(* Logix 5000 AddOnInstructionDefinition export Banner_Q90R2KU_Param_v4; software revision 33.00 *)

TYPE Banner_IOL_Port_v4 :   // UDT that has all of the data items necessary to communicate with a specific Port on a IO-Link Master
STRUCT
   Port_Controlled : INT;   // Each bit represents a port on an IO-Link Master. Set to 1 to tell AOI to control that port.
   Port_Activate : INT;   // Each bit represents a port on an IO-Link Master. When ON that port will process any commands in queue.
   Port_Read : INT;   // Each bit represents a port on an IO-Link Master. Used to determine when device AOI has requested a Read command.
   Port_Write : INT;   // Each bit represents a port on an IO-Link Master. Used to determine when device AOI has requested a Write command.
   Port_RW_Complete : INT;   // Each bit represents a port on an IO-Link Master. Tells device AOI that Read or Write request has been completed.
   Port_Device_Read : INT;
   Data_Transfer : SINT[190];   // Array to transfer data from IO-Master to device AOIs.
END_STRUCT
END_TYPE

TYPE Banner_Q90R2KR_AO1_Config_v4 :
STRUCT
   Output_Type : INT;   // 0=4-20mA, 128=0-10V, 129=0.5-4.5V.
   Measurement : SINT;   // 0=Distance or Y, 1=Velocity
   Loss_of_Signal : SINT;   // 0=Hold, 1=Low, 2=High
   Average : INT;   // 0=1, 1=2, 2=4, 3=8, 4=16, 5=32, 6=64, 7=128
END_STRUCT
END_TYPE

TYPE Banner_Q90R2KU_ActiveSensingRange :
STRUCT
   Detection_Area : SINT;   // 0=Radial, 1=Rectangular
   Radial_Min_Active_Sensing_Distance : DINT;
   Radial_Max_Active_Sensing_Distance : DINT;
   Rectangular_Min_Active_Sensing_Y : DINT;
   Rectangular_Max_Active_Sensing_Y : DINT;
   Velocity_Filter : INT;   // 0=All target velocities, 1=Dynamic targets only, 2=Approaching targets only, 3=Receding targets only, 4=custom
   Min_Velocity : DINT;
   Max_Velocity : DINT;
   Velocity_Hysteresis : DINT;
END_STRUCT
END_TYPE

TYPE Banner_Q90R2KU_AO1_Detection_Area :
STRUCT
   Peak_Select_Mode : SINT;   // 0=First Peak, 1=Strongest Peak
   Radial_Beam_Angle_SP1 : INT;
   Radial_Beam_Angle_SP2 : INT;
   Radial_Beam_Angle_Hysteresis : INT;
   Rectangular_X_SP1 : DINT;
   Rectangular_X_SP2 : DINT;
   Rectangular_X_Hysteresis : DINT;
END_STRUCT
END_TYPE

TYPE Banner_Q90R2KU_AO1_Setpoints_v4 :
STRUCT
   Radial_Distance_SP1 : DINT;
   Radial_Distance_SP2 : DINT;
   Rectangular_Y_SP1 : DINT;
   Rectangular_Y_SP2 : DINT;
   Velocity_SP1 : DINT;
   Velocity_SP2 : DINT;
END_STRUCT
END_TYPE

TYPE Banner_Q90R2KU_Config_v4 :
STRUCT
   Response_Speed : SINT;   // 0 = Fast, 1 = Medium, 2 = Slow
   Detection_Sensitivity : SINT;   // 0=High, 1=Standard
   LEDs_Disabled : SINT;   // 0=Enabled, 1=Standard
   Output_Polarity : SINT;   // 0=NPN, 1=PNP
   PD_Measurement : SINT;   // 0=Radial, 1=Rectangular
   Remote_Input_Mode : SINT;   // 0=Disabled, 1=Teach
   Amplitude_Threshold : DINT;   // 100 to 100000
   Limit_Filter_Enabled : SINT;   // 0=Disabled, 1=Enabled
   Limit_Filter_Positive_Hold_Time : DINT;   // 50 to 3600000
   Limit_Filter_Negative_Hold_Time : DINT;   // 50 to 3600000
   Limit_Filter_Positive_Distance : DINT;   // 0 to 1000
   Limit_Filter_Negative_Distance : DINT;   // 0 to 1000
   Primary_Output_Mode : SINT;   // 0=Independent Output, 1=Complementary Output, 2=Pulse Frequency Output
END_STRUCT
END_TYPE

TYPE Banner_Q90R2KU_Detection_Area :
STRUCT
   Peak_Select_Mode : SINT;   // 0=First Peak, 1=Strongest Peak
   Radial_Beam_Angle_SP1 : INT;
   Radial_Beam_Angle_SP2 : INT;
   Radial_Beam_Angle_Hysteresis : INT;
   Rectangular_X_SP1 : DINT;
   Rectangular_X_SP2 : DINT;
   Rectangular_X_Hysteresis : DINT;
END_STRUCT
END_TYPE

TYPE Banner_Q90R2KU_Direct_v4 :
STRUCT
   Master_Cycle_Time : INT;
   Min_Cycle_Time : INT;
   M_Sequence_Capability : INT;
   IO_Link_Version_ID : INT;
   Process_Data_Input_Length : INT;
   Process_Data_Output_Length : INT;
   Combined_Vendor_ID : DINT;   // IO-Link Vendor ID
   Vendor_ID1 : INT;
   Vendor_ID2 : INT;
   Combined_Device_ID : DINT;   // IO-Link Device ID
   Device_ID1 : INT;
   Device_ID2 : INT;
   Device_ID3 : INT;
END_STRUCT
END_TYPE

TYPE Banner_Q90R2KU_Pulse :
STRUCT
   Measurement : SINT;   // 0=Distance, 1=Velocity
   Frequency_SP1 : DINT;   // 100 to 600 Hz
   Frequency_SP2 : DINT;   // 100 to 600 Hz
   Loss_of_Signal : SINT;   // 0=Hold, 1=Low, 2=High
   Radial_Distance_SP1 : DINT;
   Radial_Distance_SP2 : DINT;
   Rectangular_Y_SP1 : DINT;
   Rectangular_Y_SP2 : DINT;
   Velocity_SP1 : DINT;
   Velocity_SP2 : DINT;
END_STRUCT
END_TYPE

TYPE Banner_Q90R2KU_RD_v4 :   // UDT that stores the Read Data for a Q90R Analog.
STRUCT
   Direct : Banner_Q90R2KU_Direct_v4;
   Serial_Number : STRING;
   Teach_State : SINT;
   SP1_TP1 : SINT;
   SP1_TP2 : SINT;
   SP2_TP1 : SINT;
   SP2_TP2 : SINT;
   Status : Banner_Q90R2KU_Status_v4;
   All_Time_Run_Time : DINT;   // Read only counter that tracks the total time sensor has been running since manufacture. Value in Hours.
END_STRUCT
END_TYPE

TYPE Banner_Q90R2KU_SSC1_Configuration :
STRUCT
   Switch_Point_Logic : SINT;   // 0=LO, 1=DO
   Distance_or_Y_Setpoint_Mode : SINT;   // 1=Switch Mode/Single Point Mode, 2=Window Mode
END_STRUCT
END_TYPE

TYPE Banner_Q90R2KU_SSC1_Setpoints :
STRUCT
   Radial_Distance_SP1 : DINT;
   Radial_Distance_SP2 : DINT;
   Radial_Distance_Hysteresis : DINT;
   Rectangular_Y_SP1 : DINT;
   Rectangular_Y_SP2 : DINT;
   Rectangular_Y_Hysteresis : DINT;
END_STRUCT
END_TYPE

TYPE Banner_Q90R2KU_Status_v4 :
STRUCT
   SSC1_State : SINT;   // 0=Inactive, 1=Active
   SSC1_Stability : SINT;   // 0=No target, 1=Marginal target, 2=Strong target
   SSC1_Distance_or_X : DINT;
   SSC1_Beam_Angle_or_Y : DINT;
   SSC1_Velocity : DINT;
   SSC1_Signal_Strength : INT;
   AO1_State : SINT;   // 0=Inactive, 1=Active
   AO1_Stability : SINT;   // 0=No target, 1=Marginal target, 2=Strong target
   AO1_Distance_or_X : DINT;
   AO1_Beam_Angle_or_Y : DINT;
   AO1_Velocity : DINT;
   AO1_Signal_Strength : INT;
   Fault_Status : SINT;   // 0=No fault present, 1=fault present
   Analog_Output_Value : DINT;
   Temperature : DINT;
   Last_Taught_Temperature : DINT;
END_STRUCT
END_TYPE

TYPE Banner_Q90R2KU_v4 :   // All of the parameters for a Q90R2 Analog.
STRUCT
   Initial_Global_Read : BOOL;   // Determines if all of the IO-Link data has been read into the PLC yet
   Command : INT;   // Value placed in here will activate a read or write to a specifc IO-Link Index
   Read : Banner_Q90R2KU_RD_v4;   // Read Only Data
   Write : Banner_Q90R2KU_WD_v4;   // Write Data
   Archive : Banner_Q90R2KU_WD_v4;   // Archive Data
   Reset : BOOL;   // Resets AOI. This will force a complete parameter read of the sensor.
END_STRUCT
END_TYPE

TYPE Banner_Q90R2KU_Vendor_Specific_Config_v4 :
STRUCT
   Delay_On : DINT;
   Delay_Off : DINT;
   Radial_Distance_Window_Size : DINT;   // This will set the size of the distance window after a teach.
   Radial_Distance_User_Teach_Offset : DINT;   // Distance offset applied to taught switch position.
   Radial_Reserved_Window_Size : DINT;   // This will set the size of the beam-angle window after a teach.
   Radial_Reserved_User_Teach_Offset : DINT;
   Rectangular_Reserved_Window_Size : DINT;
   Rectangular_Reserved_User_Teach_Offset : DINT;
   Rectangular_Y_Window_Size : DINT;
   Rectangular_Y_User_Teach_Offset : DINT;
END_STRUCT
END_TYPE

TYPE Banner_Q90R2KU_WD_v4 :   // UDT that stores the Write Data for a Q90R2KU.
STRUCT
   System_Command : INT;   // See IODD file for list of commands that can be activated via the System Command interface
   Teach_Selection : SINT;   // 0 = Default, 1 = BDC1, 192 = AO1
   Config : Banner_Q90R2KU_Config_v4;
   SSC1_Vendor_Config : Banner_Q90R2KU_Vendor_Specific_Config_v4;
   Resettable_Run_Time : DINT;
   AO1_Setpoints : Banner_Q90R2KU_AO1_Setpoints_v4;
   AO1_Config : Banner_Q90R2KR_AO1_Config_v4;
   All_Time_Run_Time_Event_Time : DINT;
   Resettable_Run_Time_Event_Time : DINT;
   Active_Sensing_Range : Banner_Q90R2KU_ActiveSensingRange;
   SSC1_Config : Banner_Q90R2KU_SSC1_Configuration;
   SSC1_Setpoints : Banner_Q90R2KU_SSC1_Setpoints;
   SSC1_Detection : Banner_Q90R2KU_Detection_Area;
   AO1_Detection : Banner_Q90R2KU_AO1_Detection_Area;
   Pulse : Banner_Q90R2KU_Pulse;
END_STRUCT
END_TYPE

ADD_ON_INSTRUCTION Banner_Q90R2KU_Param_v4   (* revision 4.1, vendor Banner Engineering *)
// AOI to read and write parameter data to an IO-Link Q90R2 Analog.
VAR_IN_OUT
   Q90RKU : Banner_Q90R2KU_v4; {required}
   Port_Data : Banner_IOL_Port_v4; {required}
END_VAR
VAR_INPUT
   Port : DINT; {required}
END_VAR
VAR
   Local_Control : DINT; {access None}
   Global_Read_Command_Value : INT; {access None}
   Global_Write_Command_Value : INT; {access None}
   Command_Being_Processed : BOOL; {access None}
   Update_Archive : BOOL; {access None}
   Index_Write_Inprocess : DINT; {access None}
   Index_Write_Control : DINT; {access None}
   Inprocess_Index : DINT; {access None}
END_VAR

ROUTINE Logic   (* ladder *)
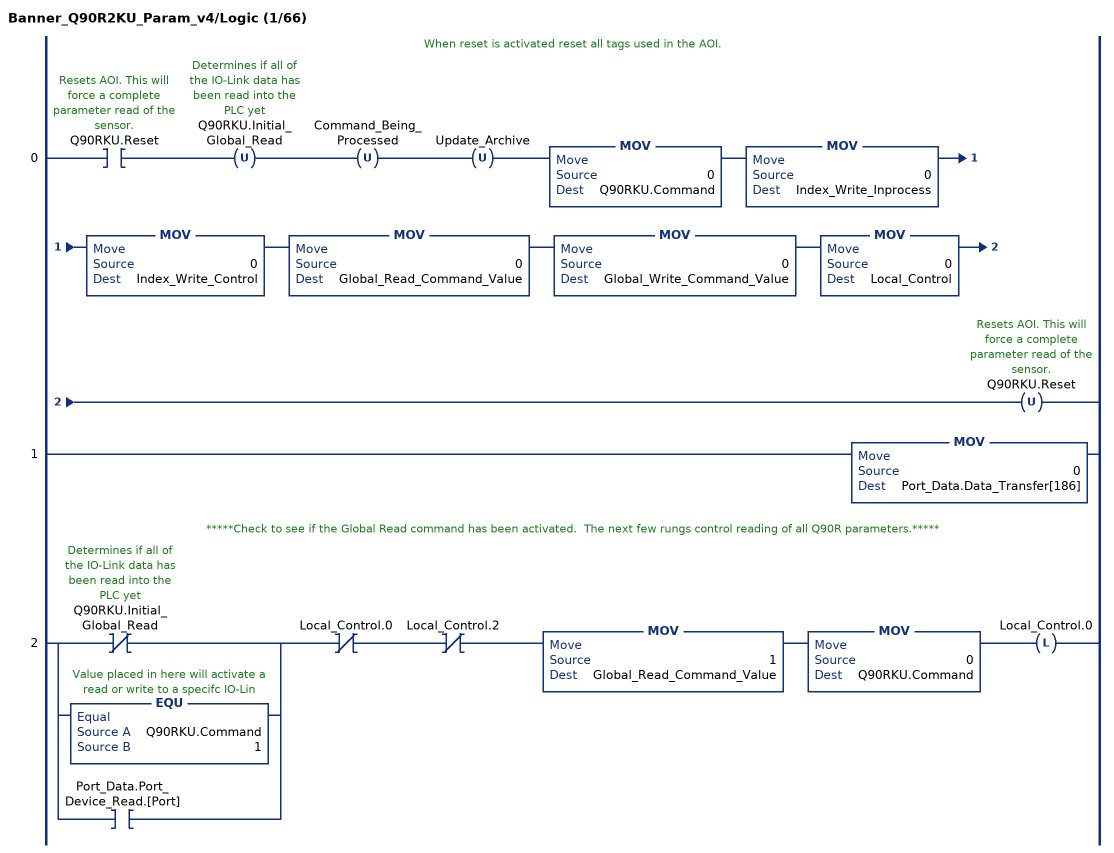
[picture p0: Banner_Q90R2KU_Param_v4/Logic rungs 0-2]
   // When reset is activated reset all tags used in the AOI.
   0: XIC(Q90RKU.Reset)OTU(Q90RKU.Initial_Global_Read)OTU(Command_Being_Processed)OTU(Update_Archive)MOV(0,Q90RKU.Command)MOV(0,Index_Write_Inprocess)MOV(0,Index_Write_Control)MOV(0,Global_Read_Command_Value)MOV(0,Global_Write_Command_Value)MOV(0,Local_Control)OTU(Q90RKU.Reset);
   1: MOV(0,Port_Data.Data_Transfer[186]);
   // *****Check to see if the Global Read command has been activated.  The next few rungs control reading of all Q90R parameters.*****
   2: [XIO(Q90RKU.Initial_Global_Read) ,EQU(Q90RKU.Command,1) ,XIC(Port_Data.Port_Device_Read.[Port]) ]XIO(Local_Control.0)XIO(Local_Control.2)MOV(1,Global_Read_Command_Value)MOV(0,Q90RKU.Command)OTL(Local_Control.0);
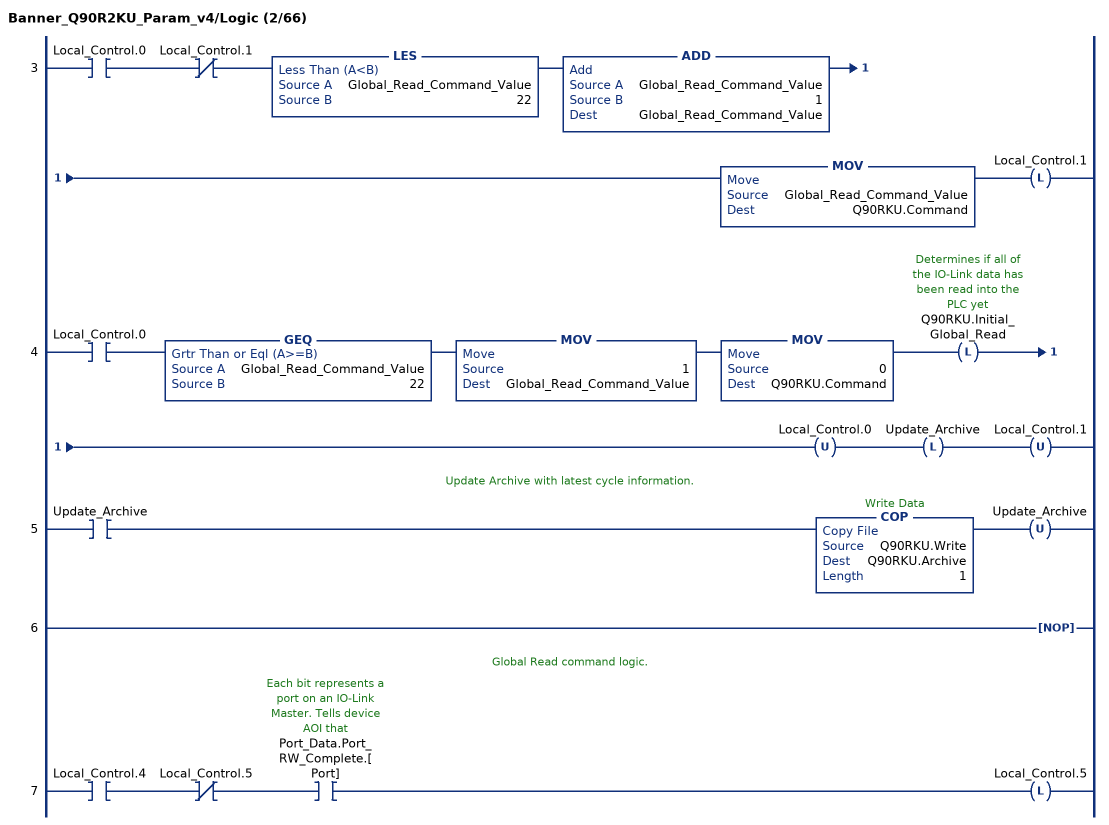
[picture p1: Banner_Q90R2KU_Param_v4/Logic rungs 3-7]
   3: XIC(Local_Control.0)XIO(Local_Control.1)LES(Global_Read_Command_Value,22)ADD(Global_Read_Command_Value,1,Global_Read_Command_Value)MOV(Global_Read_Command_Value,Q90RKU.Command)OTL(Local_Control.1);
   4: XIC(Local_Control.0)GEQ(Global_Read_Command_Value,22)MOV(1,Global_Read_Command_Value)MOV(0,Q90RKU.Command)OTL(Q90RKU.Initial_Global_Read)OTU(Local_Control.0)OTL(Update_Archive)OTU(Local_Control.1);
   // Update Archive with latest cycle information.
   5: XIC(Update_Archive)COP(Q90RKU.Write,Q90RKU.Archive,1)OTU(Update_Archive);
   6: NOP();
   // Global Read command logic.
   7: XIC(Local_Control.4)XIO(Local_Control.5)XIC(Port_Data.Port_RW_Complete.[Port])OTL(Local_Control.5);
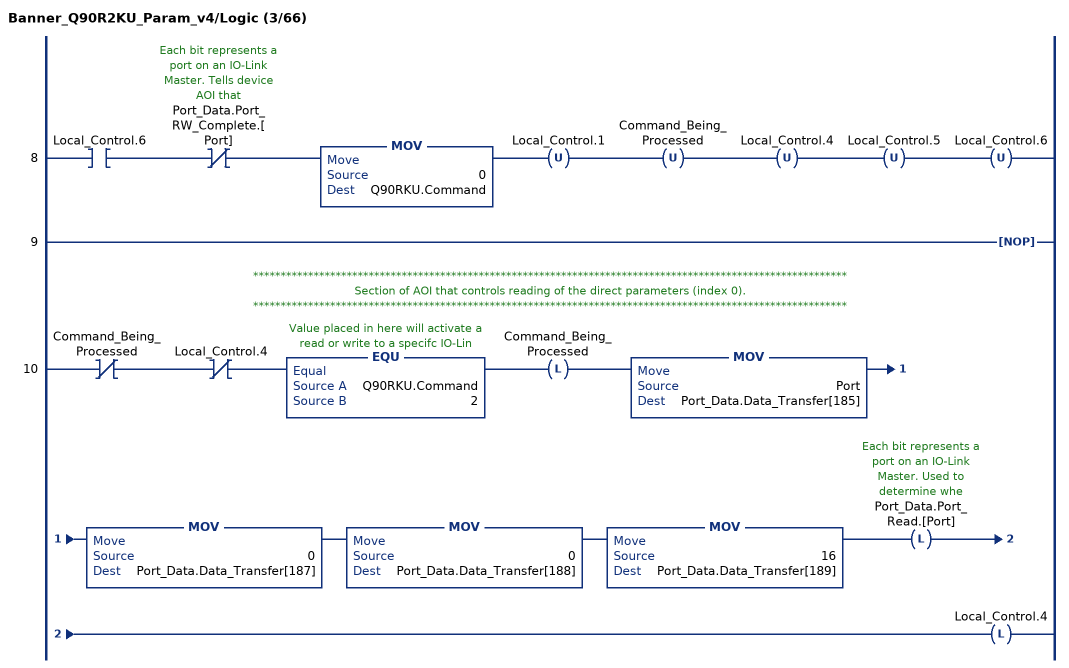
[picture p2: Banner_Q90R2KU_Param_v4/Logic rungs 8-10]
   8: XIC(Local_Control.6)XIO(Port_Data.Port_RW_Complete.[Port])MOV(0,Q90RKU.Command)OTU(Local_Control.1)OTU(Command_Being_Processed)OTU(Local_Control.4)OTU(Local_Control.5)OTU(Local_Control.6);
   9: NOP();
   // ************************************************************************************************************
   // Section of AOI that controls reading of the direct parameters (index 0).
   // ************************************************************************************************************
   10: XIO(Command_Being_Processed)XIO(Local_Control.4)EQU(Q90RKU.Command,2)OTL(Command_Being_Processed)MOV(Port,Port_Data.Data_Transfer[185])MOV(0,Port_Data.Data_Transfer[187])MOV(0,Port_Data.Data_Transfer[188])MOV(16,Port_Data.Data_Transfer[189])OTL(Port_Data.Port_Read.[Port])OTL(Local_Control.4);
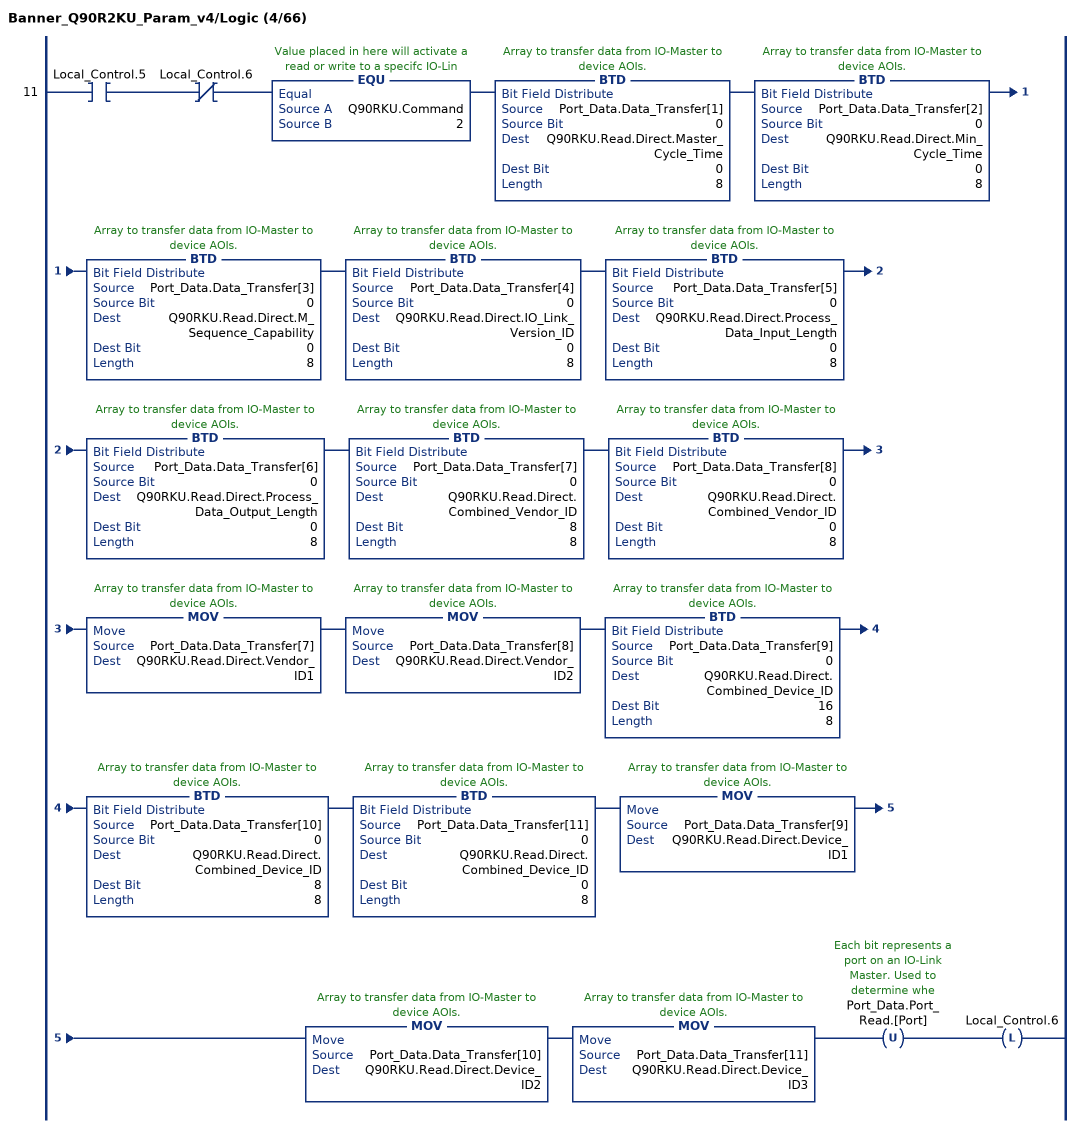
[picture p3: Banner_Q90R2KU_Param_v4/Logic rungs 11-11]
   11: XIC(Local_Control.5)XIO(Local_Control.6)EQU(Q90RKU.Command,2)BTD(Port_Data.Data_Transfer[1],0,Q90RKU.Read.Direct.Master_Cycle_Time,0,8)BTD(Port_Data.Data_Transfer[2],0,Q90RKU.Read.Direct.Min_Cycle_Time,0,8)BTD(Port_Data.Data_Transfer[3],0,Q90RKU.Read.Direct.M_Sequence_Capability,0,8)BTD(Port_Data.Data_Transfer[4],0,Q90RKU.Read.Direct.IO_Link_Version_ID,0,8)BTD(Port_Data.Data_Transfer[5],0,Q90RKU.Read.Direct.Process_Data_Input_Length,0,8)BTD(Port_Data.Data_Transfer[6],0,Q90RKU.Read.Direct.Process_Data_Output_Length,0,8)BTD(Port_Data.Data_Transfer[7],0,Q90RKU.Read.Direct.Combined_Vendor_ID,8,8)BTD(Port_Data.Data_Transfer[8],0,Q90RKU.Read.Direct.Combined_Vendor_ID,0,8)MOV(Port_Data.Data_Transfer[7],Q90RKU.Read.Direct.Vendor_ID1)MOV(Port_Data.Data_Transfer[8],Q90RKU.Read.Direct.Vendor_ID2)BTD(Port_Data.Data_Transfer[9],0,Q90RKU.Read.Direct.Combined_Device_ID,16,8)BTD(Port_Data.Data_Transfer[10],0,Q90RKU.Read.Direct.Combined_Device_ID,8,8)BTD(Port_Data.Data_Transfer[11],0,Q90RKU.Read.Direct.Combined_Device_ID,0,8)MOV(Port_Data.Data_Transfer[9],Q90RKU.Read.Direct.Device_ID1)MOV(Port_Data.Data_Transfer[10],Q90RKU.Read.Direct.Device_ID2)MOV(Port_Data.Data_Transfer[11],Q90RKU.Read.Direct.Device_ID3)OTU(Port_Data.Port_Read.[Port])OTL(Local_Control.6);
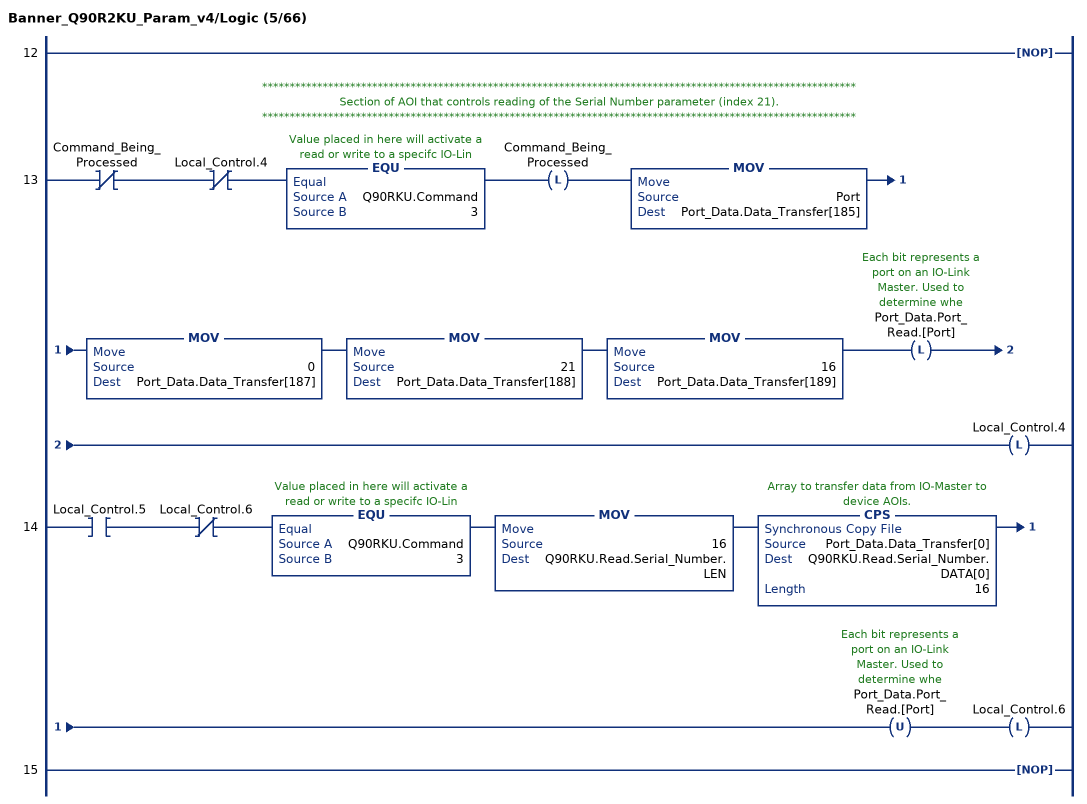
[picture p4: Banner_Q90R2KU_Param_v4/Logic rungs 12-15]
   12: NOP();
   // ************************************************************************************************************
   // Section of AOI that controls reading of the Serial Number parameter (index 21).
   // ************************************************************************************************************
   13: XIO(Command_Being_Processed)XIO(Local_Control.4)EQU(Q90RKU.Command,3)OTL(Command_Being_Processed)MOV(Port,Port_Data.Data_Transfer[185])MOV(0,Port_Data.Data_Transfer[187])MOV(21,Port_Data.Data_Transfer[188])MOV(16,Port_Data.Data_Transfer[189])OTL(Port_Data.Port_Read.[Port])OTL(Local_Control.4);
   14: XIC(Local_Control.5)XIO(Local_Control.6)EQU(Q90RKU.Command,3)MOV(16,Q90RKU.Read.Serial_Number.LEN)CPS(Port_Data.Data_Transfer[0],Q90RKU.Read.Serial_Number.DATA[0],16)OTU(Port_Data.Port_Read.[Port])OTL(Local_Control.6);
   15: NOP();
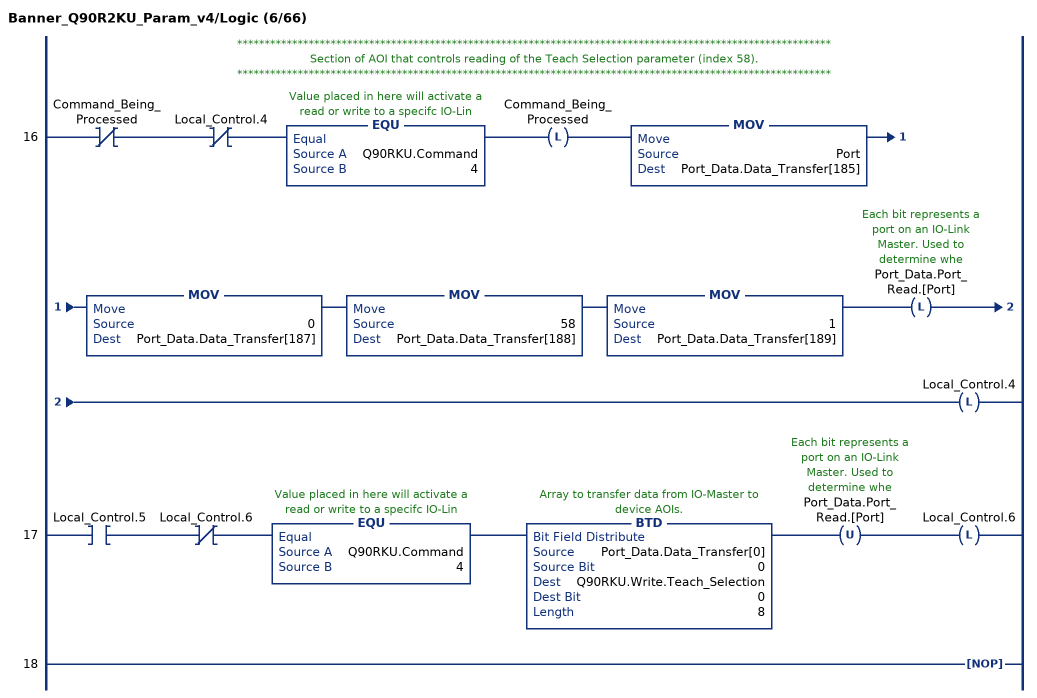
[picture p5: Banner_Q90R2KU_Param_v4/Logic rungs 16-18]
   // ************************************************************************************************************
   // Section of AOI that controls reading of the Teach Selection parameter (index 58).
   // ************************************************************************************************************
   16: XIO(Command_Being_Processed)XIO(Local_Control.4)EQU(Q90RKU.Command,4)OTL(Command_Being_Processed)MOV(Port,Port_Data.Data_Transfer[185])MOV(0,Port_Data.Data_Transfer[187])MOV(58,Port_Data.Data_Transfer[188])MOV(1,Port_Data.Data_Transfer[189])OTL(Port_Data.Port_Read.[Port])OTL(Local_Control.4);
   17: XIC(Local_Control.5)XIO(Local_Control.6)EQU(Q90RKU.Command,4)BTD(Port_Data.Data_Transfer[0],0,Q90RKU.Write.Teach_Selection,0,8)OTU(Port_Data.Port_Read.[Port])OTL(Local_Control.6);
   18: NOP();
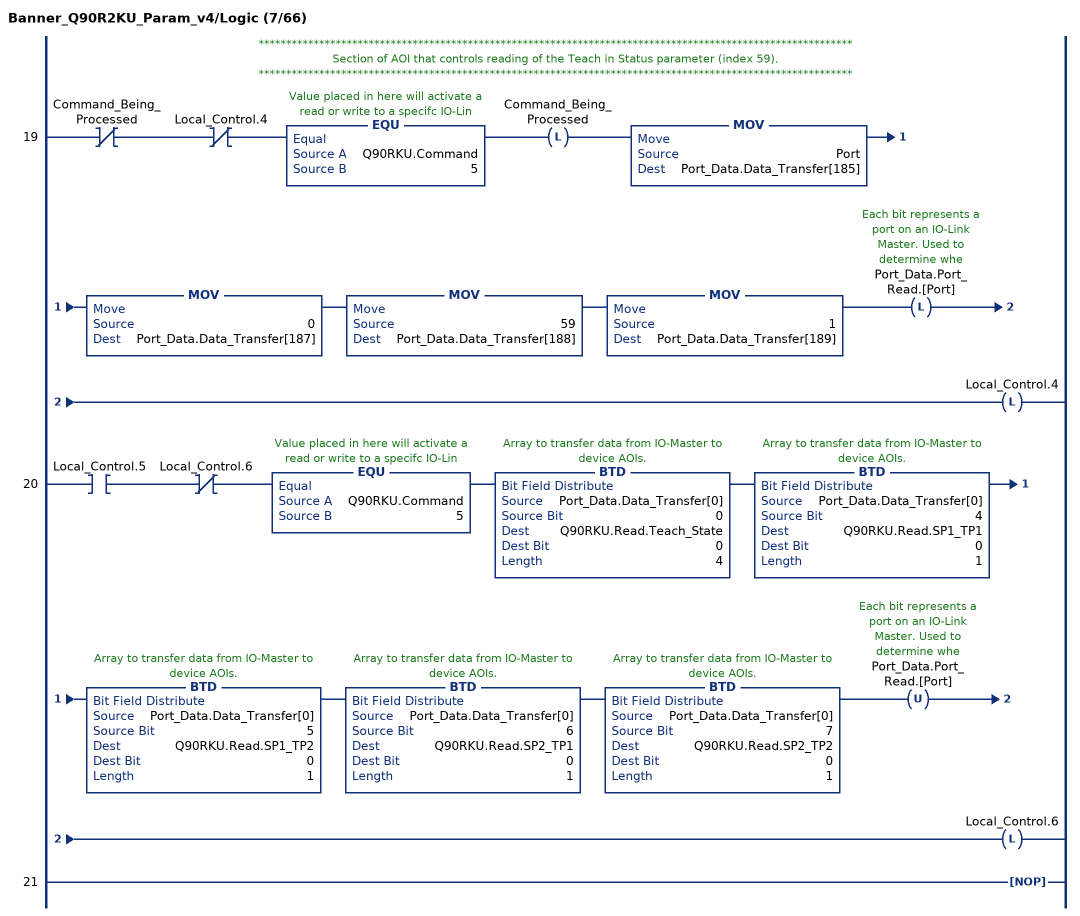
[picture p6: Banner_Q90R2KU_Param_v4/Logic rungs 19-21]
   // ************************************************************************************************************
   // Section of AOI that controls reading of the Teach in Status parameter (index 59).
   // ************************************************************************************************************
   19: XIO(Command_Being_Processed)XIO(Local_Control.4)EQU(Q90RKU.Command,5)OTL(Command_Being_Processed)MOV(Port,Port_Data.Data_Transfer[185])MOV(0,Port_Data.Data_Transfer[187])MOV(59,Port_Data.Data_Transfer[188])MOV(1,Port_Data.Data_Transfer[189])OTL(Port_Data.Port_Read.[Port])OTL(Local_Control.4);
   20: XIC(Local_Control.5)XIO(Local_Control.6)EQU(Q90RKU.Command,5)BTD(Port_Data.Data_Transfer[0],0,Q90RKU.Read.Teach_State,0,4)BTD(Port_Data.Data_Transfer[0],4,Q90RKU.Read.SP1_TP1,0,1)BTD(Port_Data.Data_Transfer[0],5,Q90RKU.Read.SP1_TP2,0,1)BTD(Port_Data.Data_Transfer[0],6,Q90RKU.Read.SP2_TP1,0,1)BTD(Port_Data.Data_Transfer[0],7,Q90RKU.Read.SP2_TP2,0,1)OTU(Port_Data.Port_Read.[Port])OTL(Local_Control.6);
   21: NOP();
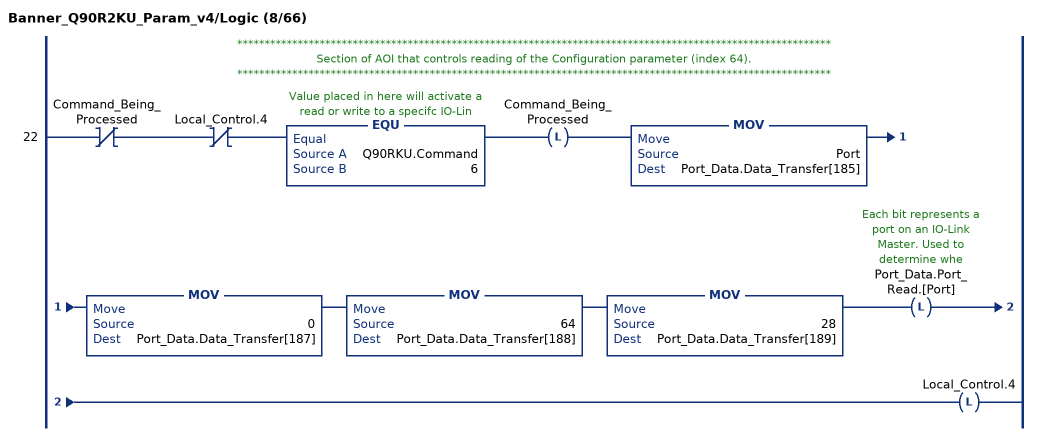
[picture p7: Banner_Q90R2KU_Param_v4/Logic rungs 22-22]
   // ************************************************************************************************************
   // Section of AOI that controls reading of the Configuration parameter (index 64).
   // ************************************************************************************************************
   22: XIO(Command_Being_Processed)XIO(Local_Control.4)EQU(Q90RKU.Command,6)OTL(Command_Being_Processed)MOV(Port,Port_Data.Data_Transfer[185])MOV(0,Port_Data.Data_Transfer[187])MOV(64,Port_Data.Data_Transfer[188])MOV(28,Port_Data.Data_Transfer[189])OTL(Port_Data.Port_Read.[Port])OTL(Local_Control.4);
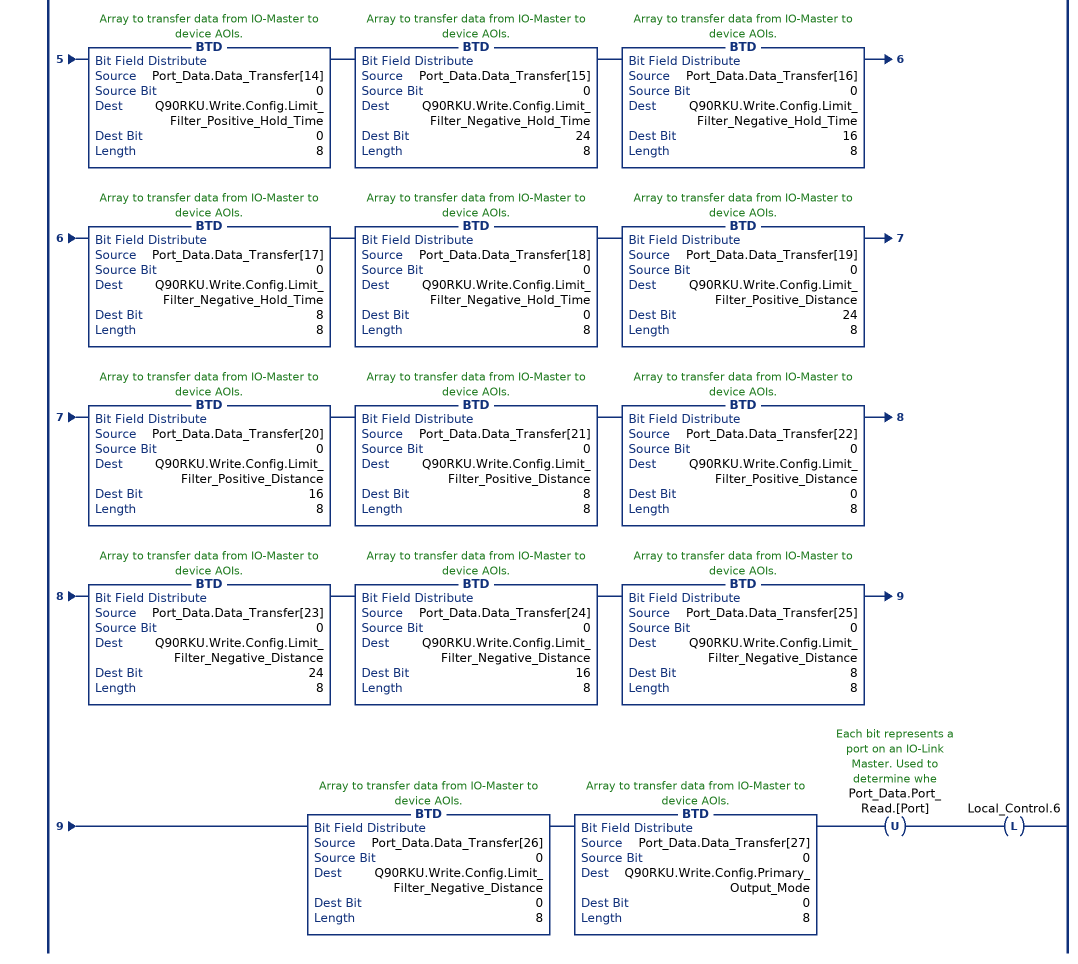
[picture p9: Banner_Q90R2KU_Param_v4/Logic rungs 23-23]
   23: XIC(Local_Control.5)XIO(Local_Control.6)EQU(Q90RKU.Command,6)BTD(Port_Data.Data_Transfer[0],0,Q90RKU.Write.Config.Response_Speed,0,8)BTD(Port_Data.Data_Transfer[1],0,Q90RKU.Write.Config.Detection_Sensitivity,0,8)BTD(Port_Data.Data_Transfer[2],0,Q90RKU.Write.Config.LEDs_Disabled,0,8)BTD(Port_Data.Data_Transfer[3],0,Q90RKU.Write.Config.Output_Polarity,0,8)BTD(Port_Data.Data_Transfer[4],0,Q90RKU.Write.Config.PD_Measurement,0,8)BTD(Port_Data.Data_Transfer[5],0,Q90RKU.Write.Config.Remote_Input_Mode,0,8)BTD(Port_Data.Data_Transfer[6],0,Q90RKU.Write.Config.Amplitude_Threshold,24,8)BTD(Port_Data.Data_Transfer[7],0,Q90RKU.Write.Config.Amplitude_Threshold,16,8)BTD(Port_Data.Data_Transfer[8],0,Q90RKU.Write.Config.Amplitude_Threshold,8,8)BTD(Port_Data.Data_Transfer[9],0,Q90RKU.Write.Config.Amplitude_Threshold,0,8)BTD(Port_Data.Data_Transfer[10],0,Q90RKU.Write.Config.Limit_Filter_Enabled,0,8)BTD(Port_Data.Data_Transfer[11],0,Q90RKU.Write.Config.Limit_Filter_Positive_Hold_Time,24,8)BTD(Port_Data.Data_Transfer[12],0,Q90RKU.Write.Config.Limit_Filter_Positive_Hold_Time,16,8)BTD(Port_Data.Data_Transfer[13],0,Q90RKU.Write.Config.Limit_Filter_Positive_Hold_Time,8,8)BTD(Port_Data.Data_Transfer[14],0,Q90RKU.Write.Config.Limit_Filter_Positive_Hold_Time,0,8)BTD(Port_Data.Data_Transfer[15],0,Q90RKU.Write.Config.Limit_Filter_Negative_Hold_Time,24,8)BTD(Port_Data.Data_Transfer[16],0,Q90RKU.Write.Config.Limit_Filter_Negative_Hold_Time,16,8)BTD(Port_Data.Data_Transfer[17],0,Q90RKU.Write.Config.Limit_Filter_Negative_Hold_Time,8,8)BTD(Port_Data.Data_Transfer[18],0,Q90RKU.Write.Config.Limit_Filter_Negative_Hold_Time,0,8)BTD(Port_Data.Data_Transfer[19],0,Q90RKU.Write.Config.Limit_Filter_Positive_Distance,24,8)BTD(Port_Data.Data_Transfer[20],0,Q90RKU.Write.Config.Limit_Filter_Positive_Distance,16,8)BTD(Port_Data.Data_Transfer[21],0,Q90RKU.Write.Config.Limit_Filter_Positive_Distance,8,8)BTD(Port_Data.Data_Transfer[22],0,Q90RKU.Write.Config.Limit_Filter_Positive_Distance,0,8)BTD(Port_Data.Data_Transfer[23],0,Q90RKU.Write.Config.Limit_Filter_Negative_Distance,24,8)BTD(Port_Data.Data_Transfer[24],0,Q90RKU.Write.Config.Limit_Filter_Negative_Distance,16,8)BTD(Port_Data.Data_Transfer[25],0,Q90RKU.Write.Config.Limit_Filter_Negative_Distance,8,8)BTD(Port_Data.Data_Transfer[26],0,Q90RKU.Write.Config.Limit_Filter_Negative_Distance,0,8)BTD(Port_Data.Data_Transfer[27],0,Q90RKU.Write.Config.Primary_Output_Mode,0,8)OTU(Port_Data.Port_Read.[Port])OTL(Local_Control.6);
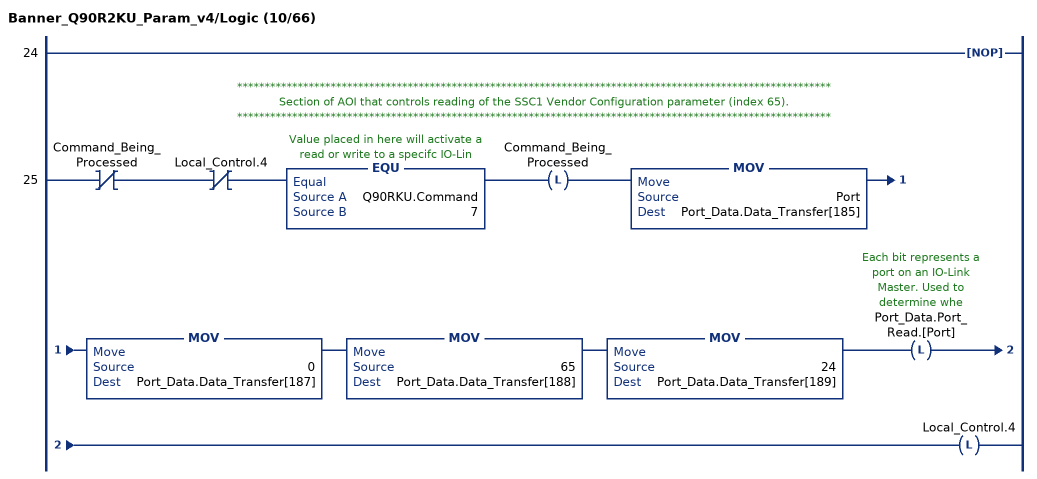
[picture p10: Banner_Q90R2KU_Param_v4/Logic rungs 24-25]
   24: NOP();
   // ************************************************************************************************************
   // Section of AOI that controls reading of the SSC1 Vendor Configuration parameter (index 65).
   // ************************************************************************************************************
   25: XIO(Command_Being_Processed)XIO(Local_Control.4)EQU(Q90RKU.Command,7)OTL(Command_Being_Processed)MOV(Port,Port_Data.Data_Transfer[185])MOV(0,Port_Data.Data_Transfer[187])MOV(65,Port_Data.Data_Transfer[188])MOV(24,Port_Data.Data_Transfer[189])OTL(Port_Data.Port_Read.[Port])OTL(Local_Control.4);
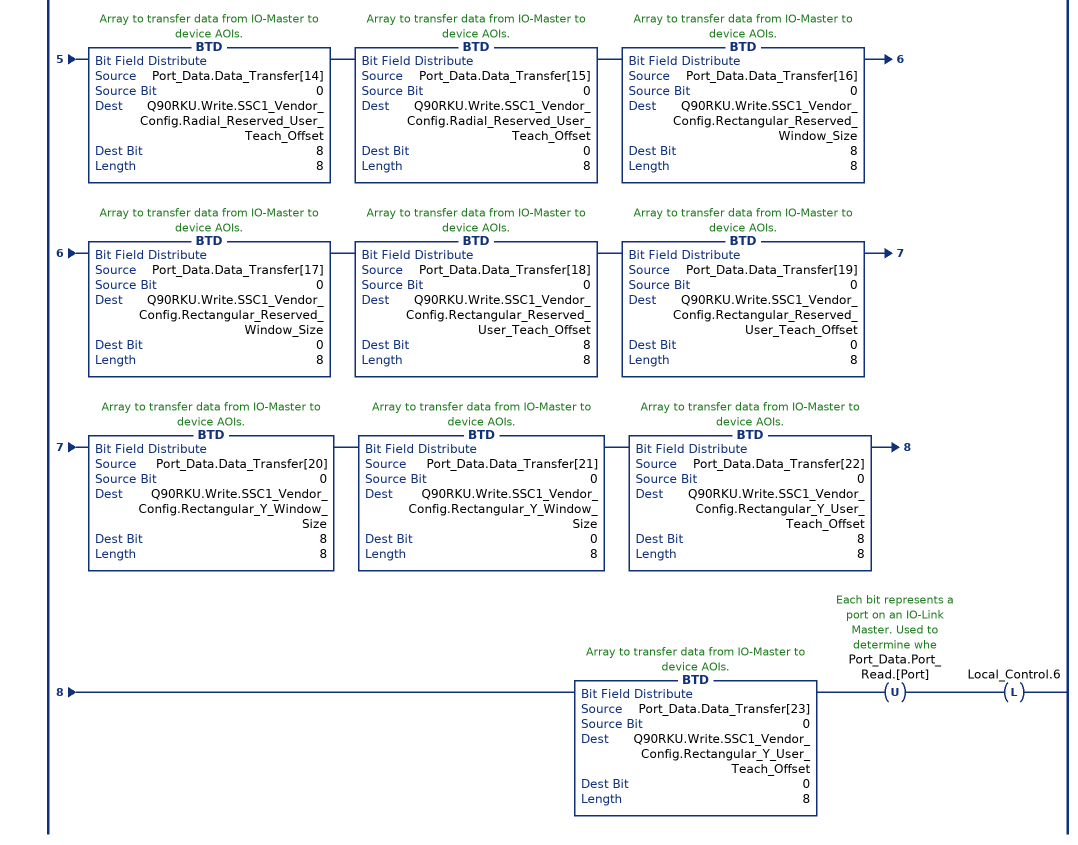
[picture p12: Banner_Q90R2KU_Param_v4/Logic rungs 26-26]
   26: XIC(Local_Control.5)XIO(Local_Control.6)EQU(Q90RKU.Command,7)BTD(Port_Data.Data_Transfer[0],0,Q90RKU.Write.SSC1_Vendor_Config.Delay_On,24,8)BTD(Port_Data.Data_Transfer[1],0,Q90RKU.Write.SSC1_Vendor_Config.Delay_On,16,8)BTD(Port_Data.Data_Transfer[2],0,Q90RKU.Write.SSC1_Vendor_Config.Delay_On,8,8)BTD(Port_Data.Data_Transfer[3],0,Q90RKU.Write.SSC1_Vendor_Config.Delay_On,0,8)BTD(Port_Data.Data_Transfer[4],0,Q90RKU.Write.SSC1_Vendor_Config.Delay_Off,24,8)BTD(Port_Data.Data_Transfer[5],0,Q90RKU.Write.SSC1_Vendor_Config.Delay_Off,16,8)BTD(Port_Data.Data_Transfer[6],0,Q90RKU.Write.SSC1_Vendor_Config.Delay_Off,8,8)BTD(Port_Data.Data_Transfer[7],0,Q90RKU.Write.SSC1_Vendor_Config.Delay_Off,0,8)BTD(Port_Data.Data_Transfer[8],0,Q90RKU.Write.SSC1_Vendor_Config.Radial_Distance_Window_Size,8,8)BTD(Port_Data.Data_Transfer[9],0,Q90RKU.Write.SSC1_Vendor_Config.Radial_Distance_Window_Size,0,8)BTD(Port_Data.Data_Transfer[10],0,Q90RKU.Write.SSC1_Vendor_Config.Radial_Distance_User_Teach_Offset,8,8)BTD(Port_Data.Data_Transfer[11],0,Q90RKU.Write.SSC1_Vendor_Config.Radial_Distance_User_Teach_Offset,0,8)BTD(Port_Data.Data_Transfer[12],0,Q90RKU.Write.SSC1_Vendor_Config.Radial_Reserved_Window_Size,8,8)BTD(Port_Data.Data_Transfer[13],0,Q90RKU.Write.SSC1_Vendor_Config.Radial_Reserved_Window_Size,0,8)BTD(Port_Data.Data_Transfer[14],0,Q90RKU.Write.SSC1_Vendor_Config.Radial_Reserved_User_Teach_Offset,8,8)BTD(Port_Data.Data_Transfer[15],0,Q90RKU.Write.SSC1_Vendor_Config.Radial_Reserved_User_Teach_Offset,0,8)BTD(Port_Data.Data_Transfer[16],0,Q90RKU.Write.SSC1_Vendor_Config.Rectangular_Reserved_Window_Size,8,8)BTD(Port_Data.Data_Transfer[17],0,Q90RKU.Write.SSC1_Vendor_Config.Rectangular_Reserved_Window_Size,0,8)BTD(Port_Data.Data_Transfer[18],0,Q90RKU.Write.SSC1_Vendor_Config.Rectangular_Reserved_User_Teach_Offset,8,8)BTD(Port_Data.Data_Transfer[19],0,Q90RKU.Write.SSC1_Vendor_Config.Rectangular_Reserved_User_Teach_Offset,0,8)BTD(Port_Data.Data_Transfer[20],0,Q90RKU.Write.SSC1_Vendor_Config.Rectangular_Y_Window_Size,8,8)BTD(Port_Data.Data_Transfer[21],0,Q90RKU.Write.SSC1_Vendor_Config.Rectangular_Y_Window_Size,0,8)BTD(Port_Data.Data_Transfer[22],0,Q90RKU.Write.SSC1_Vendor_Config.Rectangular_Y_User_Teach_Offset,8,8)BTD(Port_Data.Data_Transfer[23],0,Q90RKU.Write.SSC1_Vendor_Config.Rectangular_Y_User_Teach_Offset,0,8)OTU(Port_Data.Port_Read.[Port])OTL(Local_Control.6);
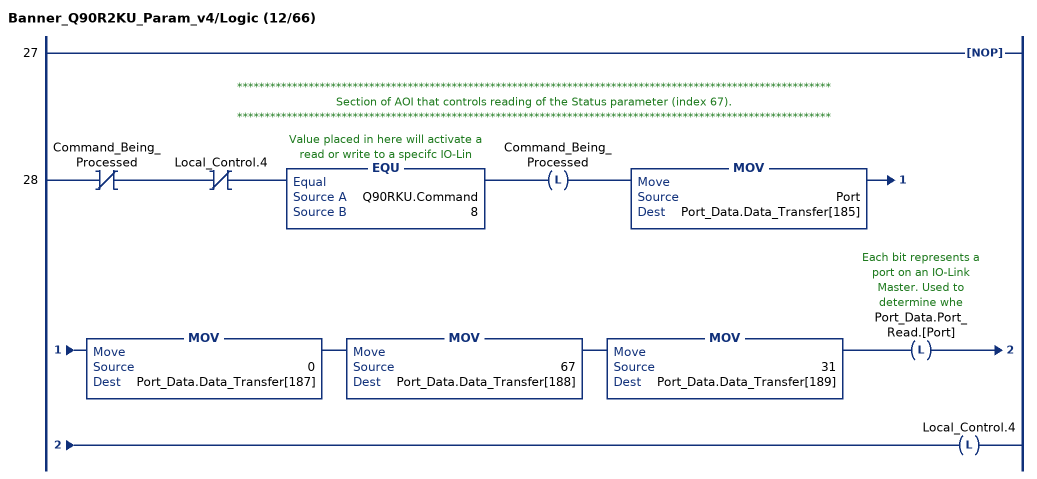
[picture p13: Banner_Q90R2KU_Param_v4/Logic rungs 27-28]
   27: NOP();
   // ************************************************************************************************************
   // Section of AOI that controls reading of the Status parameter (index 67).
   // ************************************************************************************************************
   28: XIO(Command_Being_Processed)XIO(Local_Control.4)EQU(Q90RKU.Command,8)OTL(Command_Being_Processed)MOV(Port,Port_Data.Data_Transfer[185])MOV(0,Port_Data.Data_Transfer[187])MOV(67,Port_Data.Data_Transfer[188])MOV(31,Port_Data.Data_Transfer[189])OTL(Port_Data.Port_Read.[Port])OTL(Local_Control.4);
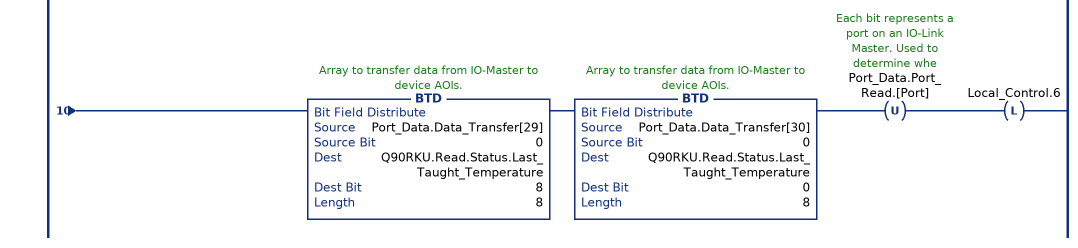
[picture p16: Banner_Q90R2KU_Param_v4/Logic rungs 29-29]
   29: XIC(Local_Control.5)XIO(Local_Control.6)EQU(Q90RKU.Command,8)BTD(Port_Data.Data_Transfer[0],0,Q90RKU.Read.Status.SSC1_State,0,8)BTD(Port_Data.Data_Transfer[1],0,Q90RKU.Read.Status.SSC1_Stability,0,8)BTD(Port_Data.Data_Transfer[2],0,Q90RKU.Read.Status.SSC1_Distance_or_X,8,8)BTD(Port_Data.Data_Transfer[3],0,Q90RKU.Read.Status.SSC1_Distance_or_X,0,8)BTD(Port_Data.Data_Transfer[4],0,Q90RKU.Read.Status.SSC1_Beam_Angle_or_Y,8,8)BTD(Port_Data.Data_Transfer[5],0,Q90RKU.Read.Status.SSC1_Beam_Angle_or_Y,0,8)BTD(Port_Data.Data_Transfer[6],0,Q90RKU.Read.Status.SSC1_Velocity,8,8)BTD(Port_Data.Data_Transfer[7],0,Q90RKU.Read.Status.SSC1_Velocity,0,8)BTD(Port_Data.Data_Transfer[8],0,Q90RKU.Read.Status.SSC1_Signal_Strength,0,8)BTD(Port_Data.Data_Transfer[9],0,Q90RKU.Read.Status.AO1_State,0,8)BTD(Port_Data.Data_Transfer[10],0,Q90RKU.Read.Status.AO1_Stability,0,8)BTD(Port_Data.Data_Transfer[11],0,Q90RKU.Read.Status.AO1_Distance_or_X,8,8)BTD(Port_Data.Data_Transfer[12],0,Q90RKU.Read.Status.AO1_Distance_or_X,0,8)BTD(Port_Data.Data_Transfer[13],0,Q90RKU.Read.Status.AO1_Beam_Angle_or_Y,8,8)BTD(Port_Data.Data_Transfer[14],0,Q90RKU.Read.Status.AO1_Beam_Angle_or_Y,0,8)BTD(Port_Data.Data_Transfer[15],0,Q90RKU.Read.Status.AO1_Velocity,8,8)BTD(Port_Data.Data_Transfer[16],0,Q90RKU.Read.Status.AO1_Velocity,0,8)BTD(Port_Data.Data_Transfer[17],0,Q90RKU.Read.Status.AO1_Signal_Strength,0,8)BTD(Port_Data.Data_Transfer[18],0,Q90RKU.Read.Status.Fault_Status,0,8)BTD(Port_Data.Data_Transfer[19],0,Q90RKU.Read.Status.Analog_Output_Value,24,8)BTD(Port_Data.Data_Transfer[20],0,Q90RKU.Read.Status.Analog_Output_Value,16,8)BTD(Port_Data.Data_Transfer[21],0,Q90RKU.Read.Status.Analog_Output_Value,8,8)BTD(Port_Data.Data_Transfer[22],0,Q90RKU.Read.Status.Analog_Output_Value,0,8)BTD(Port_Data.Data_Transfer[23],0,Q90RKU.Read.Status.Temperature,24,8)BTD(Port_Data.Data_Transfer[24],0,Q90RKU.Read.Status.Temperature,16,8)BTD(Port_Data.Data_Transfer[25],0,Q90RKU.Read.Status.Temperature,8,8)BTD(Port_Data.Data_Transfer[26],0,Q90RKU.Read.Status.Temperature,0,8)BTD(Port_Data.Data_Transfer[27],0,Q90RKU.Read.Status.Last_Taught_Temperature,24,8)BTD(Port_Data.Data_Transfer[28],0,Q90RKU.Read.Status.Last_Taught_Temperature,16,8)BTD(Port_Data.Data_Transfer[29],0,Q90RKU.Read.Status.Last_Taught_Temperature,8,8)BTD(Port_Data.Data_Transfer[30],0,Q90RKU.Read.Status.Last_Taught_Temperature,0,8)OTU(Port_Data.Port_Read.[Port])OTL(Local_Control.6);
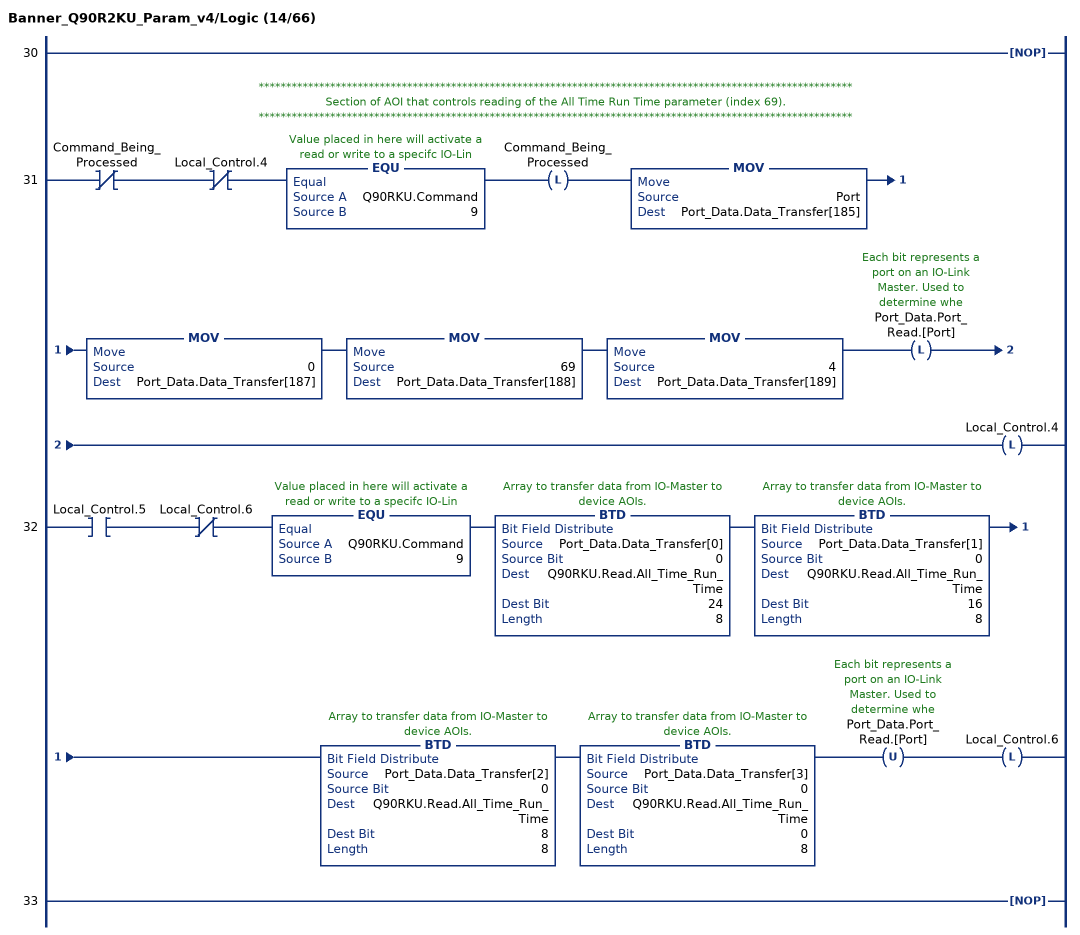
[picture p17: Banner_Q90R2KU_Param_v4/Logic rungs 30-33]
   30: NOP();
   // ************************************************************************************************************
   // Section of AOI that controls reading of the All Time Run Time parameter (index 69).
   // ************************************************************************************************************
   31: XIO(Command_Being_Processed)XIO(Local_Control.4)EQU(Q90RKU.Command,9)OTL(Command_Being_Processed)MOV(Port,Port_Data.Data_Transfer[185])MOV(0,Port_Data.Data_Transfer[187])MOV(69,Port_Data.Data_Transfer[188])MOV(4,Port_Data.Data_Transfer[189])OTL(Port_Data.Port_Read.[Port])OTL(Local_Control.4);
   32: XIC(Local_Control.5)XIO(Local_Control.6)EQU(Q90RKU.Command,9)BTD(Port_Data.Data_Transfer[0],0,Q90RKU.Read.All_Time_Run_Time,24,8)BTD(Port_Data.Data_Transfer[1],0,Q90RKU.Read.All_Time_Run_Time,16,8)BTD(Port_Data.Data_Transfer[2],0,Q90RKU.Read.All_Time_Run_Time,8,8)BTD(Port_Data.Data_Transfer[3],0,Q90RKU.Read.All_Time_Run_Time,0,8)OTU(Port_Data.Port_Read.[Port])OTL(Local_Control.6);
   33: NOP();
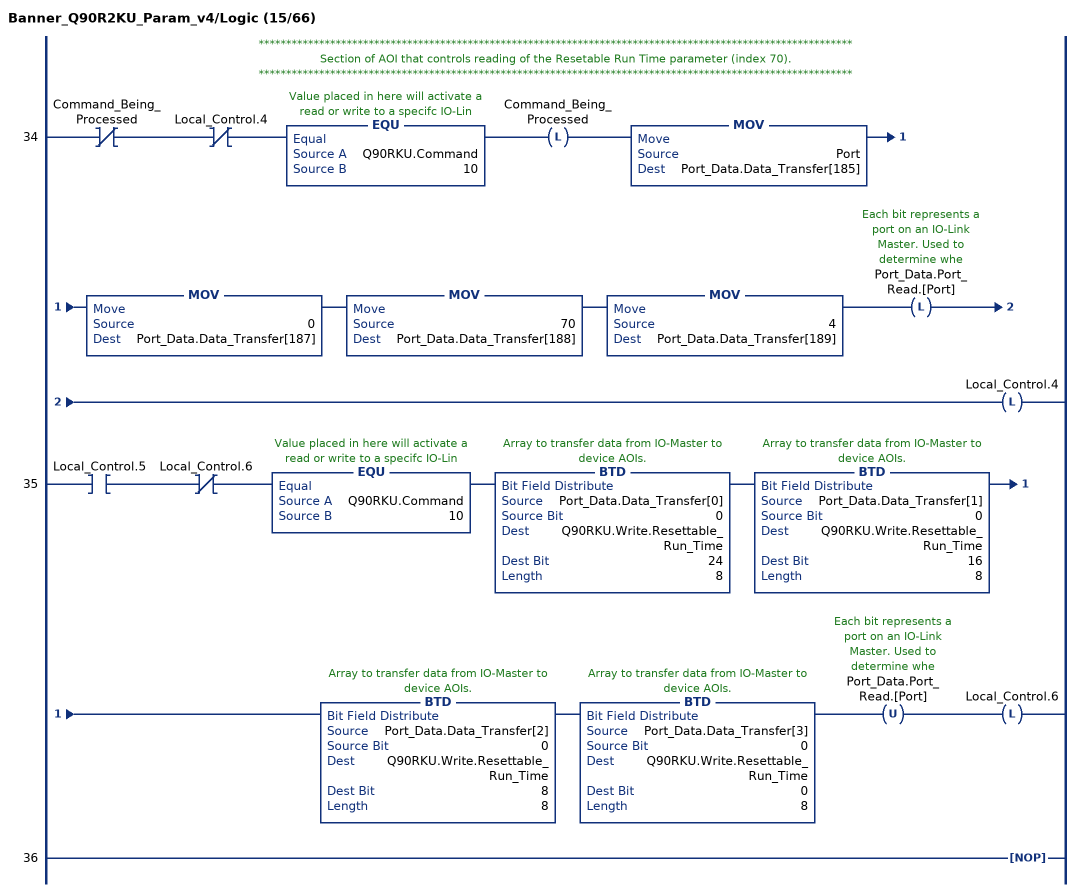
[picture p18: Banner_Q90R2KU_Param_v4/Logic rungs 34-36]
   // ************************************************************************************************************
   // Section of AOI that controls reading of the Resetable Run Time parameter (index 70).
   // ************************************************************************************************************
   34: XIO(Command_Being_Processed)XIO(Local_Control.4)EQU(Q90RKU.Command,10)OTL(Command_Being_Processed)MOV(Port,Port_Data.Data_Transfer[185])MOV(0,Port_Data.Data_Transfer[187])MOV(70,Port_Data.Data_Transfer[188])MOV(4,Port_Data.Data_Transfer[189])OTL(Port_Data.Port_Read.[Port])OTL(Local_Control.4);
   35: XIC(Local_Control.5)XIO(Local_Control.6)EQU(Q90RKU.Command,10)BTD(Port_Data.Data_Transfer[0],0,Q90RKU.Write.Resettable_Run_Time,24,8)BTD(Port_Data.Data_Transfer[1],0,Q90RKU.Write.Resettable_Run_Time,16,8)BTD(Port_Data.Data_Transfer[2],0,Q90RKU.Write.Resettable_Run_Time,8,8)BTD(Port_Data.Data_Transfer[3],0,Q90RKU.Write.Resettable_Run_Time,0,8)OTU(Port_Data.Port_Read.[Port])OTL(Local_Control.6);
   36: NOP();
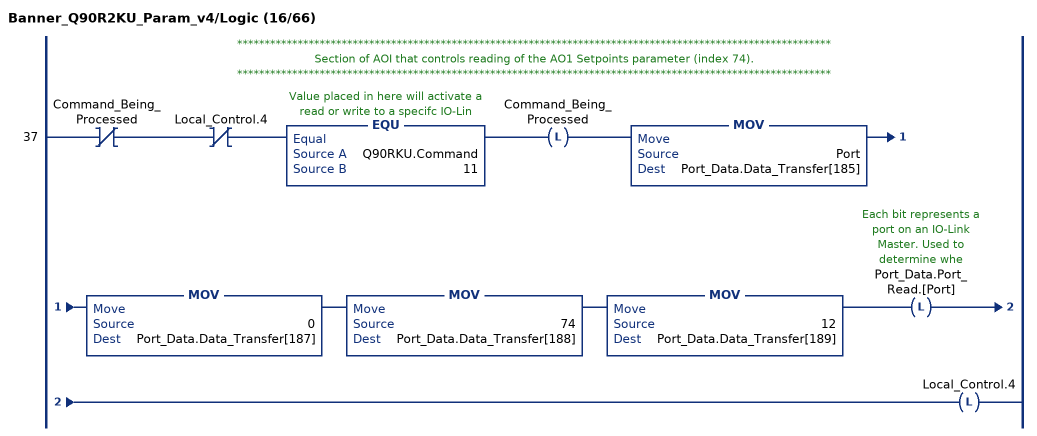
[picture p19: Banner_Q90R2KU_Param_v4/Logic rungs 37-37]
   // ************************************************************************************************************
   // Section of AOI that controls reading of the AO1 Setpoints parameter (index 74).
   // ************************************************************************************************************
   37: XIO(Command_Being_Processed)XIO(Local_Control.4)EQU(Q90RKU.Command,11)OTL(Command_Being_Processed)MOV(Port,Port_Data.Data_Transfer[185])MOV(0,Port_Data.Data_Transfer[187])MOV(74,Port_Data.Data_Transfer[188])MOV(12,Port_Data.Data_Transfer[189])OTL(Port_Data.Port_Read.[Port])OTL(Local_Control.4);
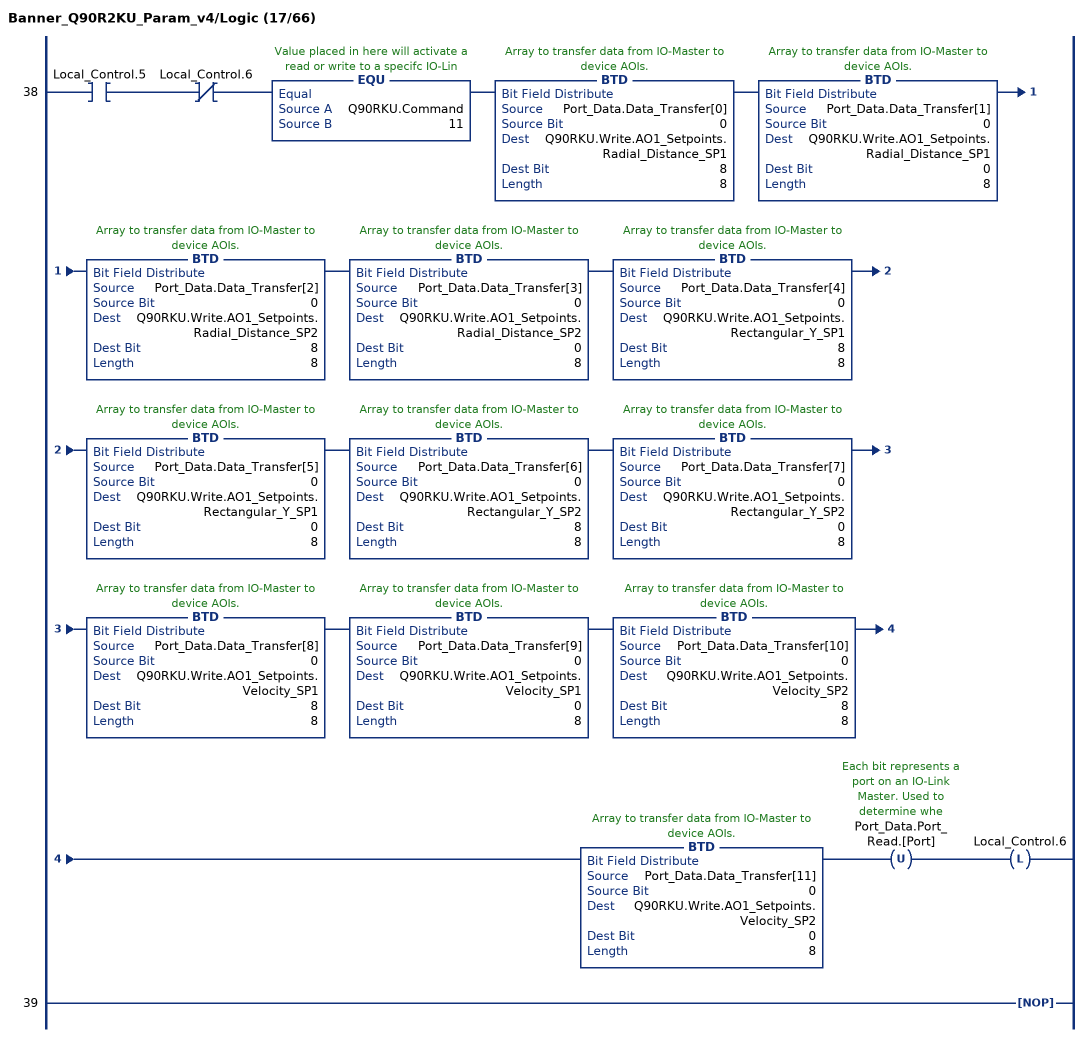
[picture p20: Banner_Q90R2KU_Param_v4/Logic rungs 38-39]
   38: XIC(Local_Control.5)XIO(Local_Control.6)EQU(Q90RKU.Command,11)BTD(Port_Data.Data_Transfer[0],0,Q90RKU.Write.AO1_Setpoints.Radial_Distance_SP1,8,8)BTD(Port_Data.Data_Transfer[1],0,Q90RKU.Write.AO1_Setpoints.Radial_Distance_SP1,0,8)BTD(Port_Data.Data_Transfer[2],0,Q90RKU.Write.AO1_Setpoints.Radial_Distance_SP2,8,8)BTD(Port_Data.Data_Transfer[3],0,Q90RKU.Write.AO1_Setpoints.Radial_Distance_SP2,0,8)BTD(Port_Data.Data_Transfer[4],0,Q90RKU.Write.AO1_Setpoints.Rectangular_Y_SP1,8,8)BTD(Port_Data.Data_Transfer[5],0,Q90RKU.Write.AO1_Setpoints.Rectangular_Y_SP1,0,8)BTD(Port_Data.Data_Transfer[6],0,Q90RKU.Write.AO1_Setpoints.Rectangular_Y_SP2,8,8)BTD(Port_Data.Data_Transfer[7],0,Q90RKU.Write.AO1_Setpoints.Rectangular_Y_SP2,0,8)BTD(Port_Data.Data_Transfer[8],0,Q90RKU.Write.AO1_Setpoints.Velocity_SP1,8,8)BTD(Port_Data.Data_Transfer[9],0,Q90RKU.Write.AO1_Setpoints.Velocity_SP1,0,8)BTD(Port_Data.Data_Transfer[10],0,Q90RKU.Write.AO1_Setpoints.Velocity_SP2,8,8)BTD(Port_Data.Data_Transfer[11],0,Q90RKU.Write.AO1_Setpoints.Velocity_SP2,0,8)OTU(Port_Data.Port_Read.[Port])OTL(Local_Control.6);
   39: NOP();
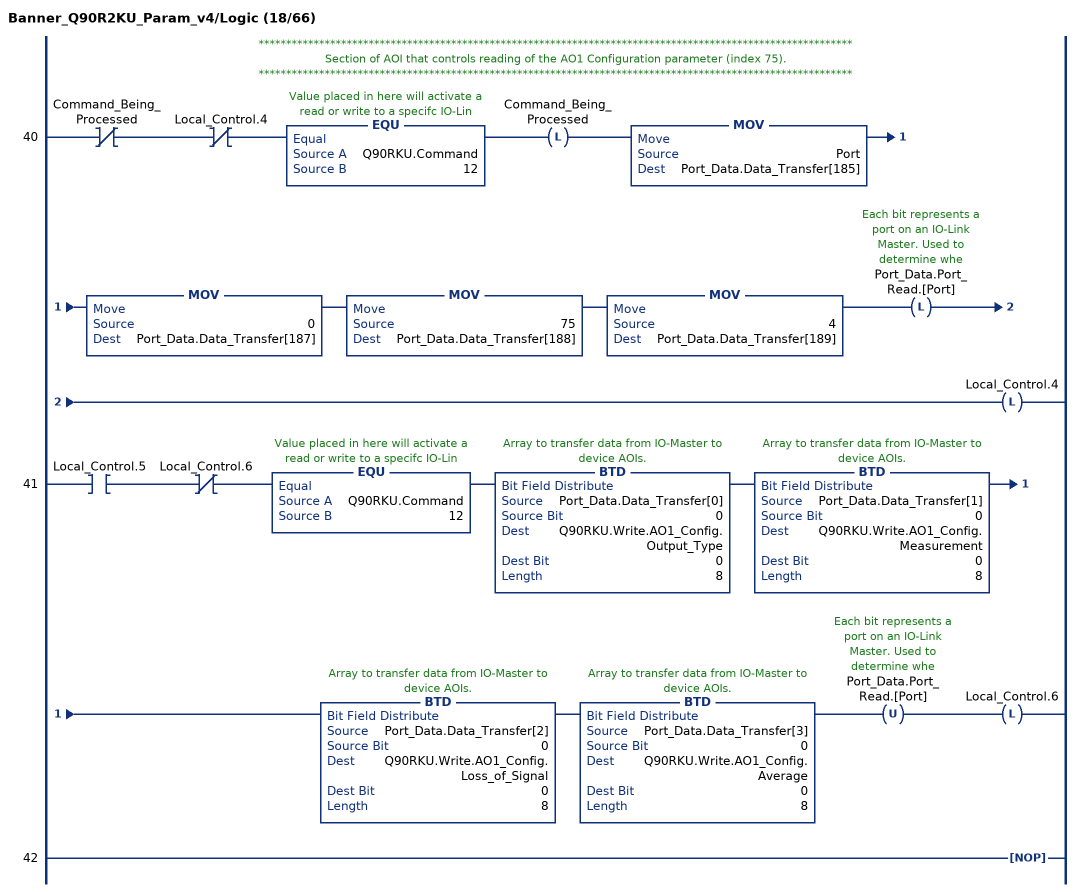
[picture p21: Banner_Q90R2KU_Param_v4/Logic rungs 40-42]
   // ************************************************************************************************************
   // Section of AOI that controls reading of the AO1 Configuration parameter (index 75).
   // ************************************************************************************************************
   40: XIO(Command_Being_Processed)XIO(Local_Control.4)EQU(Q90RKU.Command,12)OTL(Command_Being_Processed)MOV(Port,Port_Data.Data_Transfer[185])MOV(0,Port_Data.Data_Transfer[187])MOV(75,Port_Data.Data_Transfer[188])MOV(4,Port_Data.Data_Transfer[189])OTL(Port_Data.Port_Read.[Port])OTL(Local_Control.4);
   41: XIC(Local_Control.5)XIO(Local_Control.6)EQU(Q90RKU.Command,12)BTD(Port_Data.Data_Transfer[0],0,Q90RKU.Write.AO1_Config.Output_Type,0,8)BTD(Port_Data.Data_Transfer[1],0,Q90RKU.Write.AO1_Config.Measurement,0,8)BTD(Port_Data.Data_Transfer[2],0,Q90RKU.Write.AO1_Config.Loss_of_Signal,0,8)BTD(Port_Data.Data_Transfer[3],0,Q90RKU.Write.AO1_Config.Average,0,8)OTU(Port_Data.Port_Read.[Port])OTL(Local_Control.6);
   42: NOP();
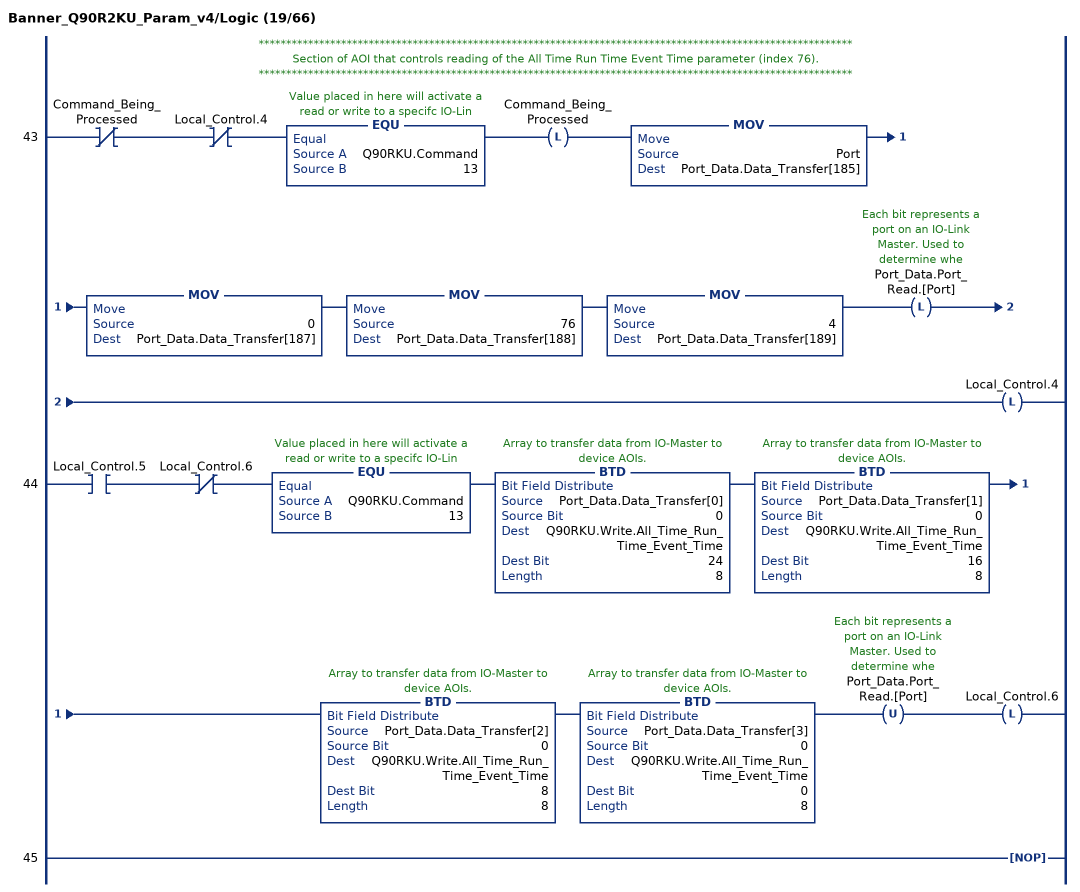
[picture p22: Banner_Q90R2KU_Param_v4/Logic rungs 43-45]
   // ************************************************************************************************************
   // Section of AOI that controls reading of the All Time Run Time Event Time parameter (index 76).
   // ************************************************************************************************************
   43: XIO(Command_Being_Processed)XIO(Local_Control.4)EQU(Q90RKU.Command,13)OTL(Command_Being_Processed)MOV(Port,Port_Data.Data_Transfer[185])MOV(0,Port_Data.Data_Transfer[187])MOV(76,Port_Data.Data_Transfer[188])MOV(4,Port_Data.Data_Transfer[189])OTL(Port_Data.Port_Read.[Port])OTL(Local_Control.4);
   44: XIC(Local_Control.5)XIO(Local_Control.6)EQU(Q90RKU.Command,13)BTD(Port_Data.Data_Transfer[0],0,Q90RKU.Write.All_Time_Run_Time_Event_Time,24,8)BTD(Port_Data.Data_Transfer[1],0,Q90RKU.Write.All_Time_Run_Time_Event_Time,16,8)BTD(Port_Data.Data_Transfer[2],0,Q90RKU.Write.All_Time_Run_Time_Event_Time,8,8)BTD(Port_Data.Data_Transfer[3],0,Q90RKU.Write.All_Time_Run_Time_Event_Time,0,8)OTU(Port_Data.Port_Read.[Port])OTL(Local_Control.6);
   45: NOP();
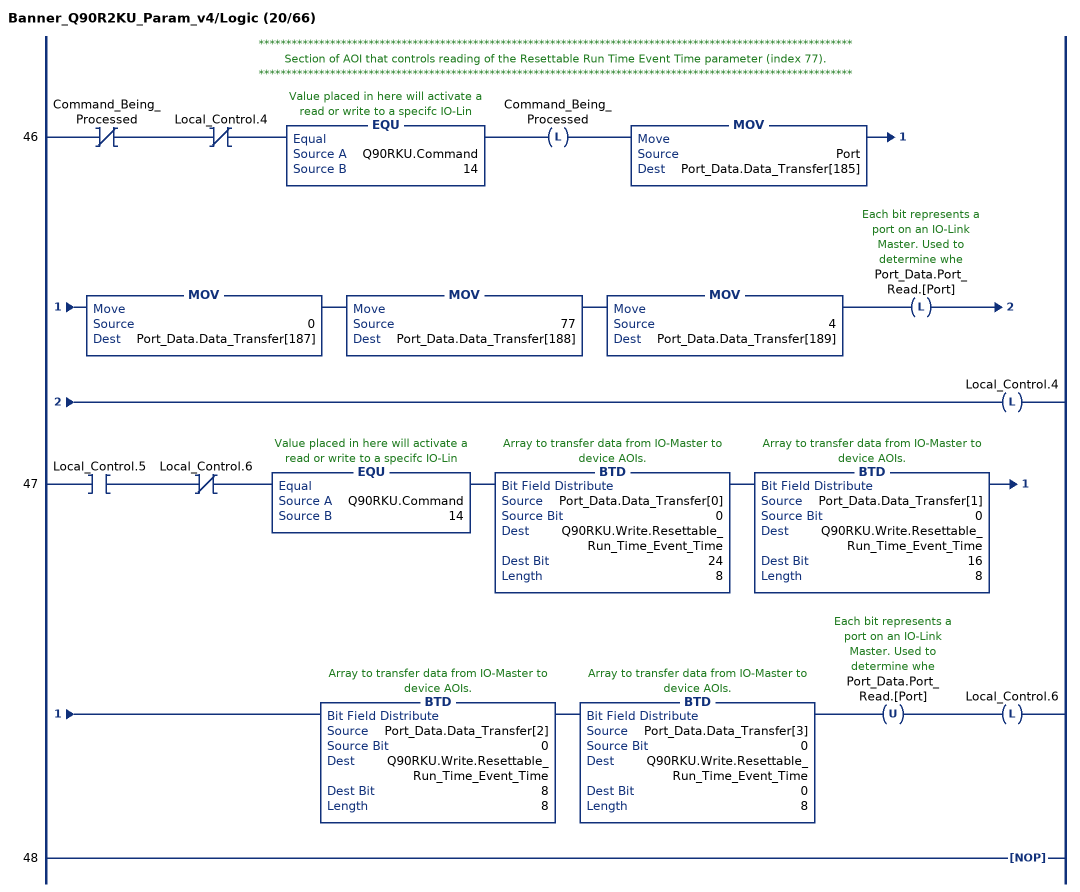
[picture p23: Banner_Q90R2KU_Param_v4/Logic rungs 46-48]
   // ************************************************************************************************************
   // Section of AOI that controls reading of the Resettable Run Time Event Time parameter (index 77).
   // ************************************************************************************************************
   46: XIO(Command_Being_Processed)XIO(Local_Control.4)EQU(Q90RKU.Command,14)OTL(Command_Being_Processed)MOV(Port,Port_Data.Data_Transfer[185])MOV(0,Port_Data.Data_Transfer[187])MOV(77,Port_Data.Data_Transfer[188])MOV(4,Port_Data.Data_Transfer[189])OTL(Port_Data.Port_Read.[Port])OTL(Local_Control.4);
   47: XIC(Local_Control.5)XIO(Local_Control.6)EQU(Q90RKU.Command,14)BTD(Port_Data.Data_Transfer[0],0,Q90RKU.Write.Resettable_Run_Time_Event_Time,24,8)BTD(Port_Data.Data_Transfer[1],0,Q90RKU.Write.Resettable_Run_Time_Event_Time,16,8)BTD(Port_Data.Data_Transfer[2],0,Q90RKU.Write.Resettable_Run_Time_Event_Time,8,8)BTD(Port_Data.Data_Transfer[3],0,Q90RKU.Write.Resettable_Run_Time_Event_Time,0,8)OTU(Port_Data.Port_Read.[Port])OTL(Local_Control.6);
   48: NOP();
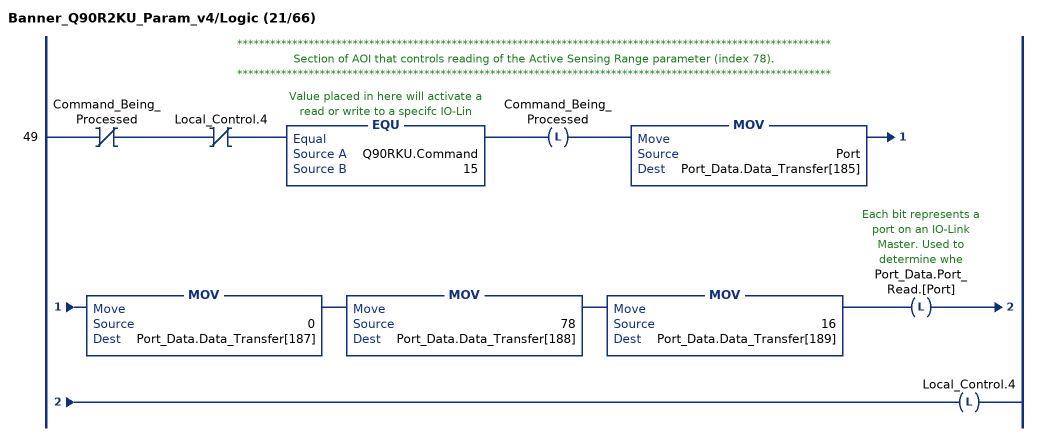
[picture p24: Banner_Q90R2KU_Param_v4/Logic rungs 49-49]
   // ************************************************************************************************************
   // Section of AOI that controls reading of the Active Sensing Range parameter (index 78).
   // ************************************************************************************************************
   49: XIO(Command_Being_Processed)XIO(Local_Control.4)EQU(Q90RKU.Command,15)OTL(Command_Being_Processed)MOV(Port,Port_Data.Data_Transfer[185])MOV(0,Port_Data.Data_Transfer[187])MOV(78,Port_Data.Data_Transfer[188])MOV(16,Port_Data.Data_Transfer[189])OTL(Port_Data.Port_Read.[Port])OTL(Local_Control.4);
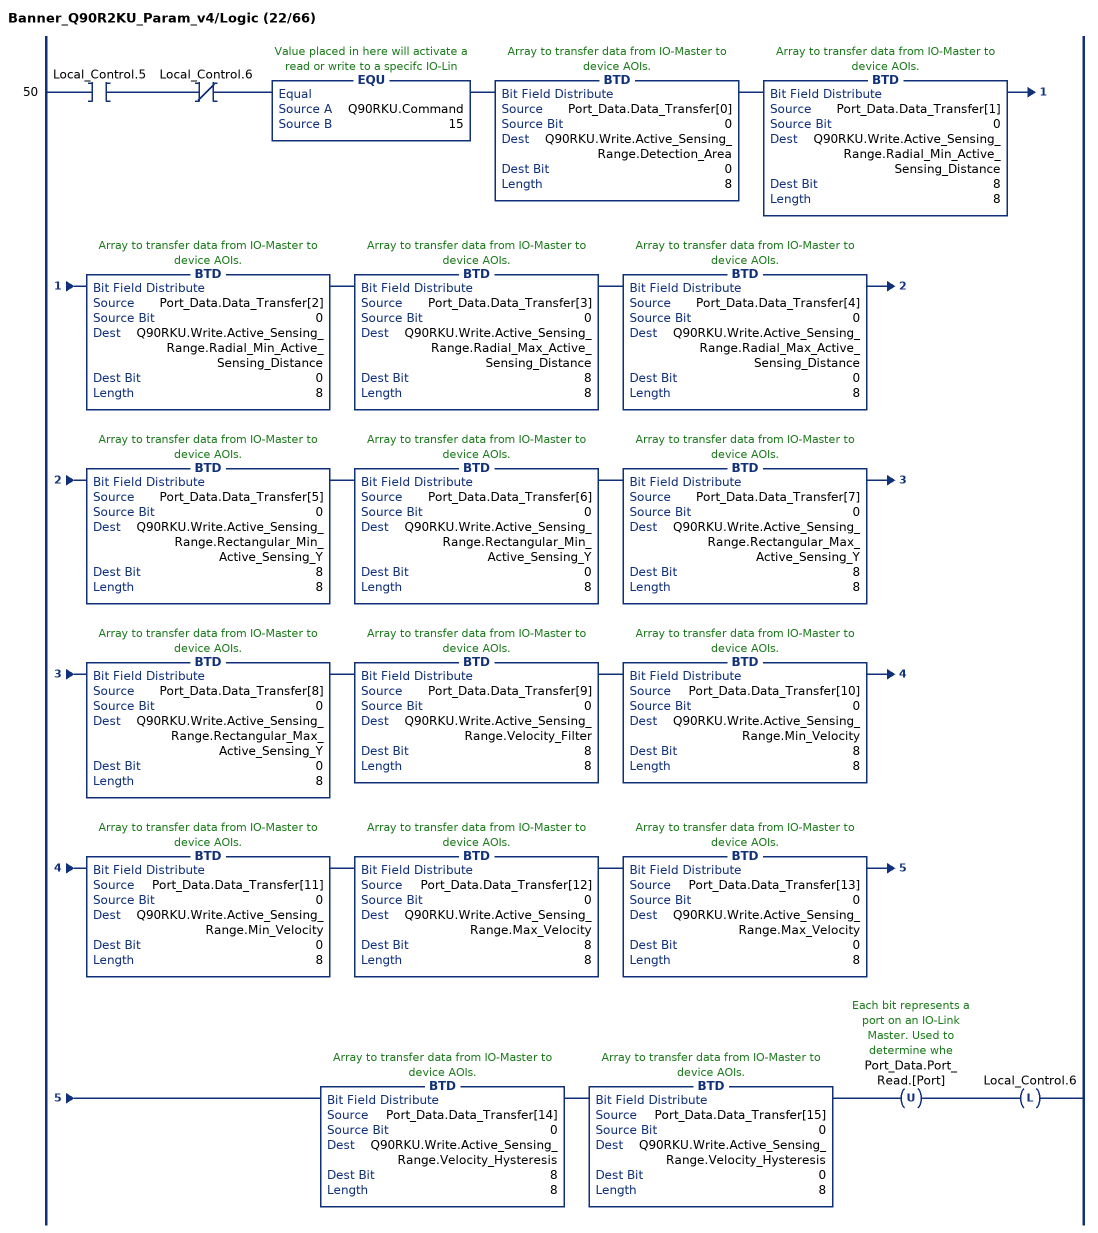
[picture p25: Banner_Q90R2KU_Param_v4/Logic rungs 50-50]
   50: XIC(Local_Control.5)XIO(Local_Control.6)EQU(Q90RKU.Command,15)BTD(Port_Data.Data_Transfer[0],0,Q90RKU.Write.Active_Sensing_Range.Detection_Area,0,8)BTD(Port_Data.Data_Transfer[1],0,Q90RKU.Write.Active_Sensing_Range.Radial_Min_Active_Sensing_Distance,8,8)BTD(Port_Data.Data_Transfer[2],0,Q90RKU.Write.Active_Sensing_Range.Radial_Min_Active_Sensing_Distance,0,8)BTD(Port_Data.Data_Transfer[3],0,Q90RKU.Write.Active_Sensing_Range.Radial_Max_Active_Sensing_Distance,8,8)BTD(Port_Data.Data_Transfer[4],0,Q90RKU.Write.Active_Sensing_Range.Radial_Max_Active_Sensing_Distance,0,8)BTD(Port_Data.Data_Transfer[5],0,Q90RKU.Write.Active_Sensing_Range.Rectangular_Min_Active_Sensing_Y,8,8)BTD(Port_Data.Data_Transfer[6],0,Q90RKU.Write.Active_Sensing_Range.Rectangular_Min_Active_Sensing_Y,0,8)BTD(Port_Data.Data_Transfer[7],0,Q90RKU.Write.Active_Sensing_Range.Rectangular_Max_Active_Sensing_Y,8,8)BTD(Port_Data.Data_Transfer[8],0,Q90RKU.Write.Active_Sensing_Range.Rectangular_Max_Active_Sensing_Y,0,8)BTD(Port_Data.Data_Transfer[9],0,Q90RKU.Write.Active_Sensing_Range.Velocity_Filter,8,8)BTD(Port_Data.Data_Transfer[10],0,Q90RKU.Write.Active_Sensing_Range.Min_Velocity,8,8)BTD(Port_Data.Data_Transfer[11],0,Q90RKU.Write.Active_Sensing_Range.Min_Velocity,0,8)BTD(Port_Data.Data_Transfer[12],0,Q90RKU.Write.Active_Sensing_Range.Max_Velocity,8,8)BTD(Port_Data.Data_Transfer[13],0,Q90RKU.Write.Active_Sensing_Range.Max_Velocity,0,8)BTD(Port_Data.Data_Transfer[14],0,Q90RKU.Write.Active_Sensing_Range.Velocity_Hysteresis,8,8)BTD(Port_Data.Data_Transfer[15],0,Q90RKU.Write.Active_Sensing_Range.Velocity_Hysteresis,0,8)OTU(Port_Data.Port_Read.[Port])OTL(Local_Control.6);
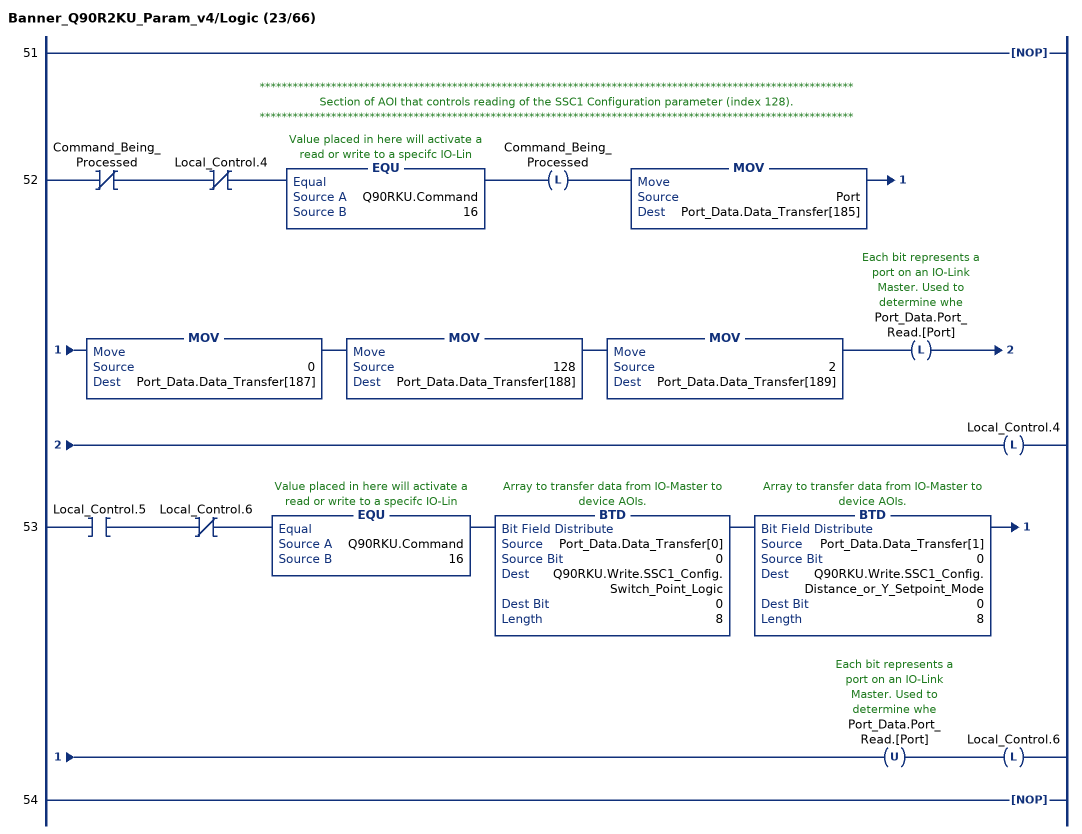
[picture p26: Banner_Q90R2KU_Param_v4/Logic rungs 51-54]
   51: NOP();
   // ************************************************************************************************************
   // Section of AOI that controls reading of the SSC1 Configuration parameter (index 128).
   // ************************************************************************************************************
   52: XIO(Command_Being_Processed)XIO(Local_Control.4)EQU(Q90RKU.Command,16)OTL(Command_Being_Processed)MOV(Port,Port_Data.Data_Transfer[185])MOV(0,Port_Data.Data_Transfer[187])MOV(128,Port_Data.Data_Transfer[188])MOV(2,Port_Data.Data_Transfer[189])OTL(Port_Data.Port_Read.[Port])OTL(Local_Control.4);
   53: XIC(Local_Control.5)XIO(Local_Control.6)EQU(Q90RKU.Command,16)BTD(Port_Data.Data_Transfer[0],0,Q90RKU.Write.SSC1_Config.Switch_Point_Logic,0,8)BTD(Port_Data.Data_Transfer[1],0,Q90RKU.Write.SSC1_Config.Distance_or_Y_Setpoint_Mode,0,8)OTU(Port_Data.Port_Read.[Port])OTL(Local_Control.6);
   54: NOP();
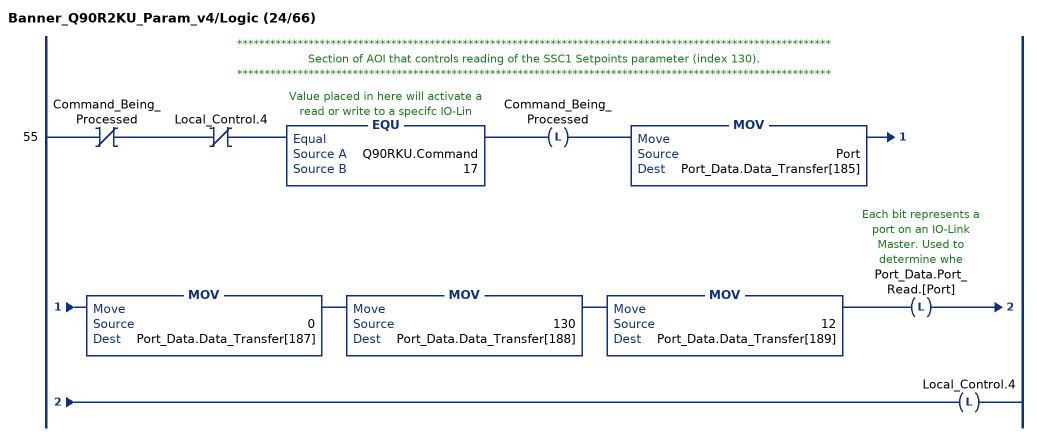
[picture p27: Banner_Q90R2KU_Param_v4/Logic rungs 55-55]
   // ************************************************************************************************************
   // Section of AOI that controls reading of the SSC1 Setpoints parameter (index 130).
   // ************************************************************************************************************
   55: XIO(Command_Being_Processed)XIO(Local_Control.4)EQU(Q90RKU.Command,17)OTL(Command_Being_Processed)MOV(Port,Port_Data.Data_Transfer[185])MOV(0,Port_Data.Data_Transfer[187])MOV(130,Port_Data.Data_Transfer[188])MOV(12,Port_Data.Data_Transfer[189])OTL(Port_Data.Port_Read.[Port])OTL(Local_Control.4);
